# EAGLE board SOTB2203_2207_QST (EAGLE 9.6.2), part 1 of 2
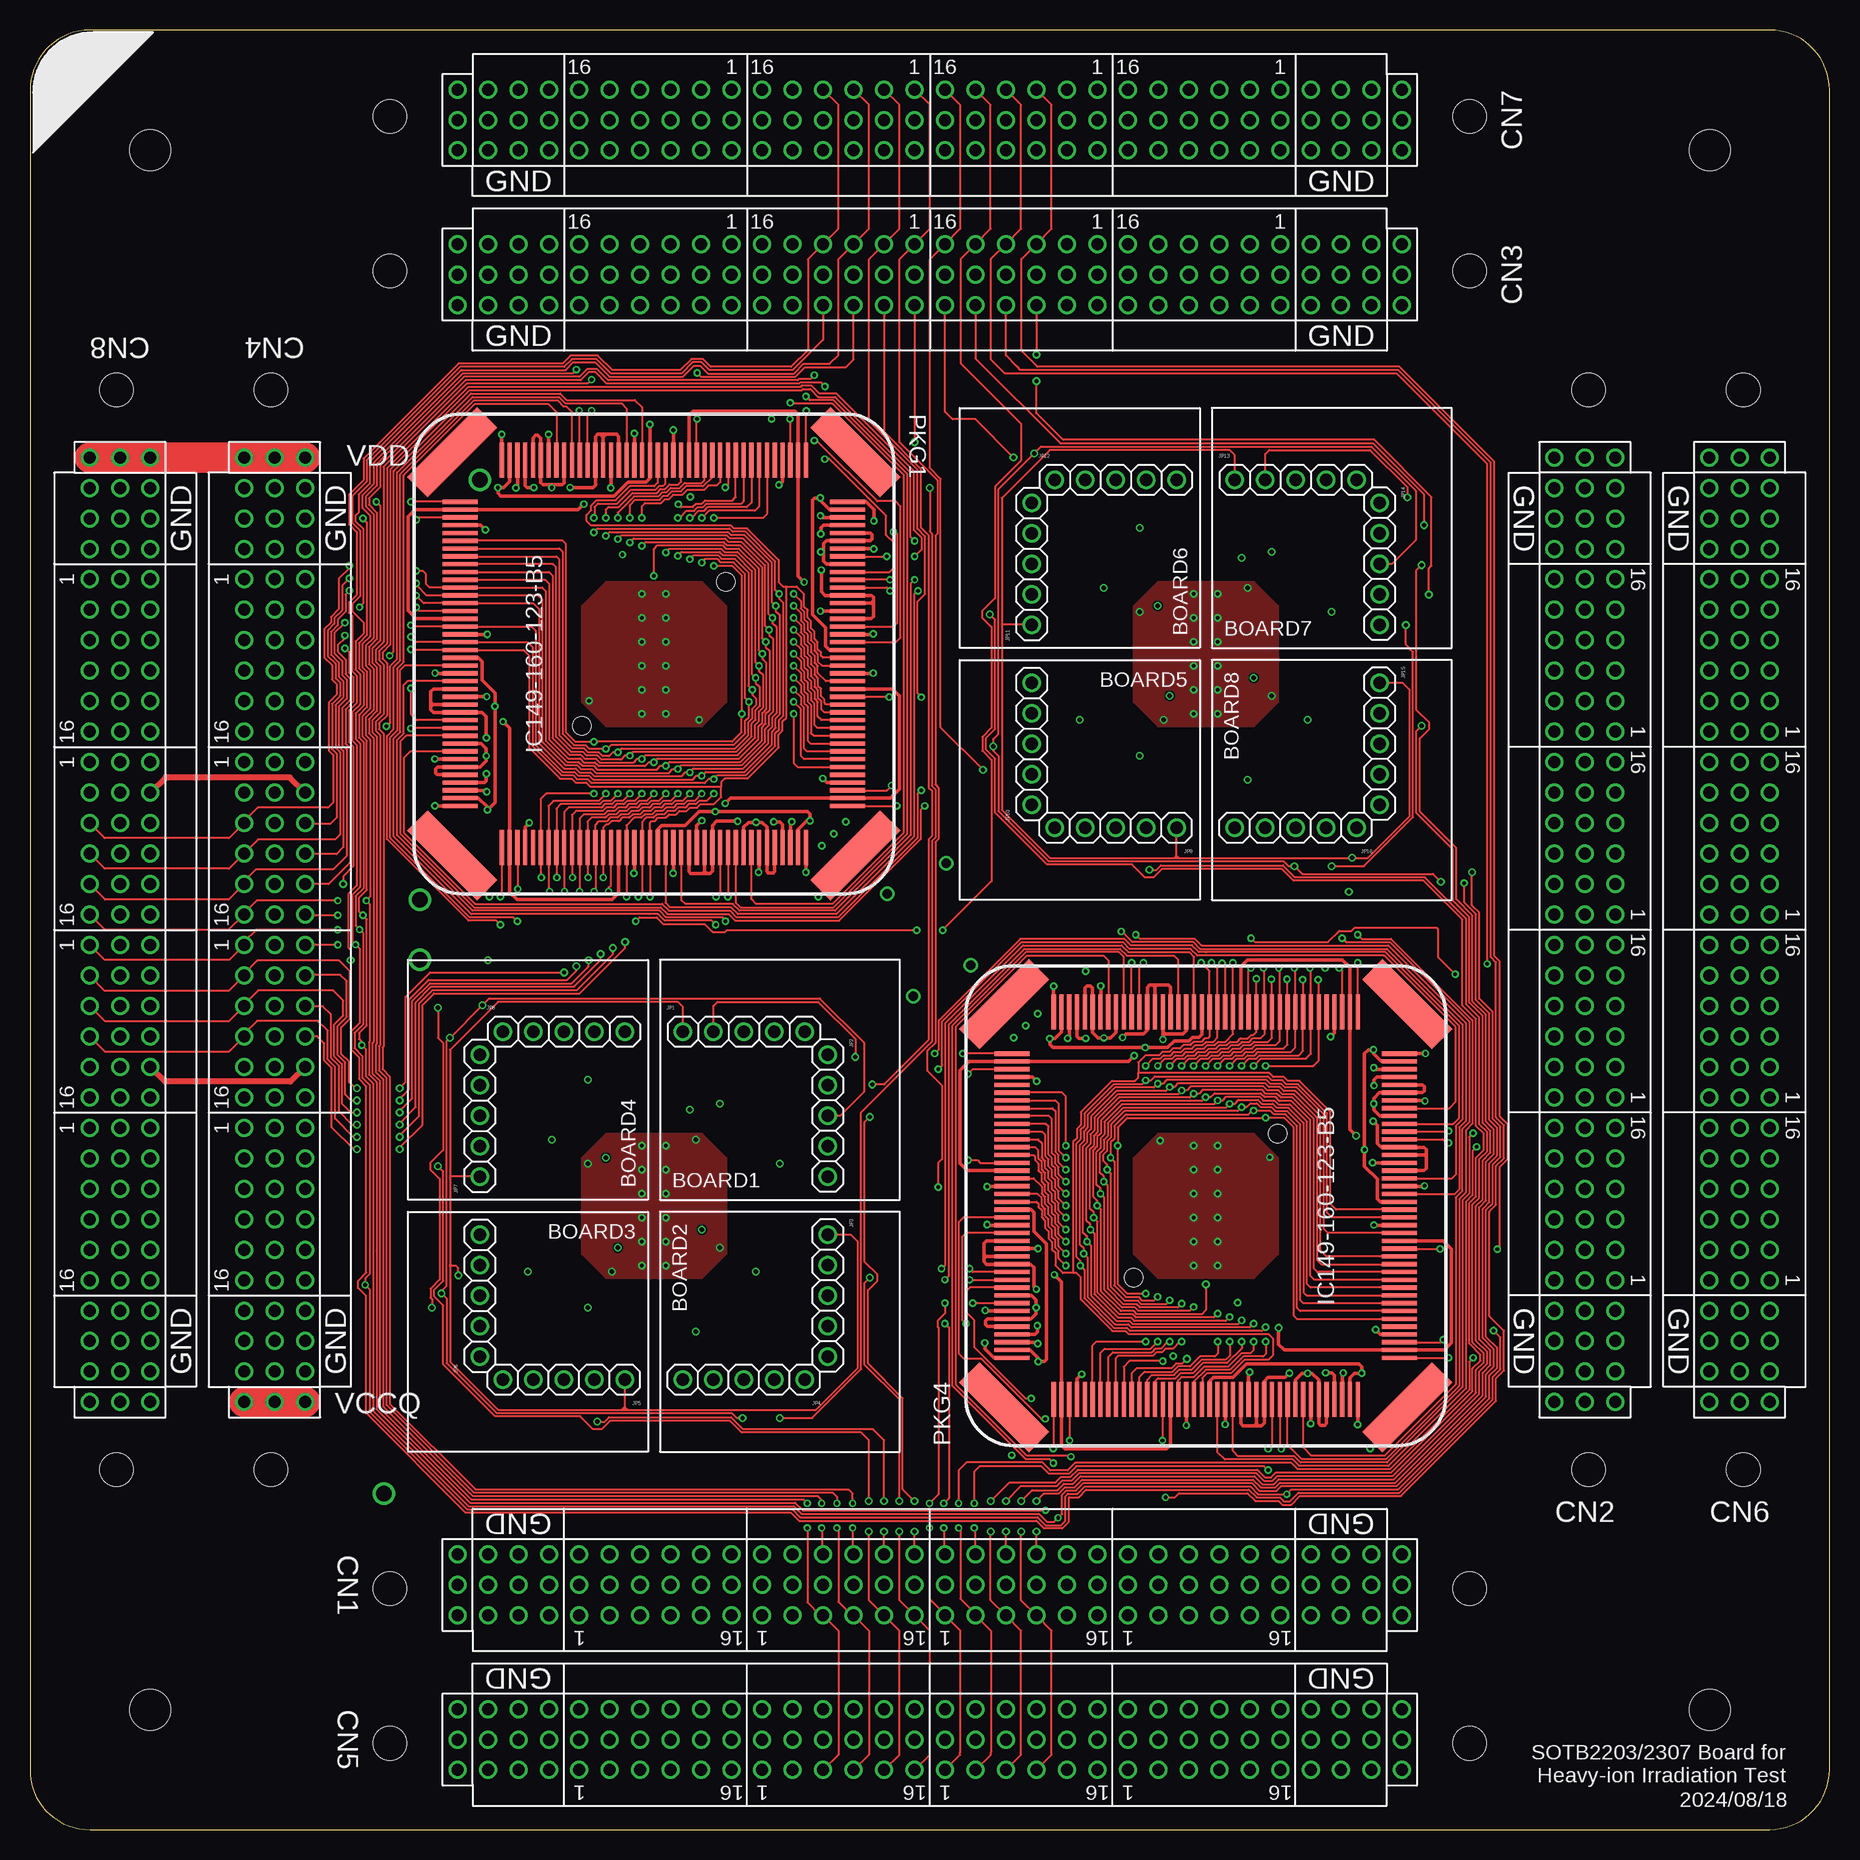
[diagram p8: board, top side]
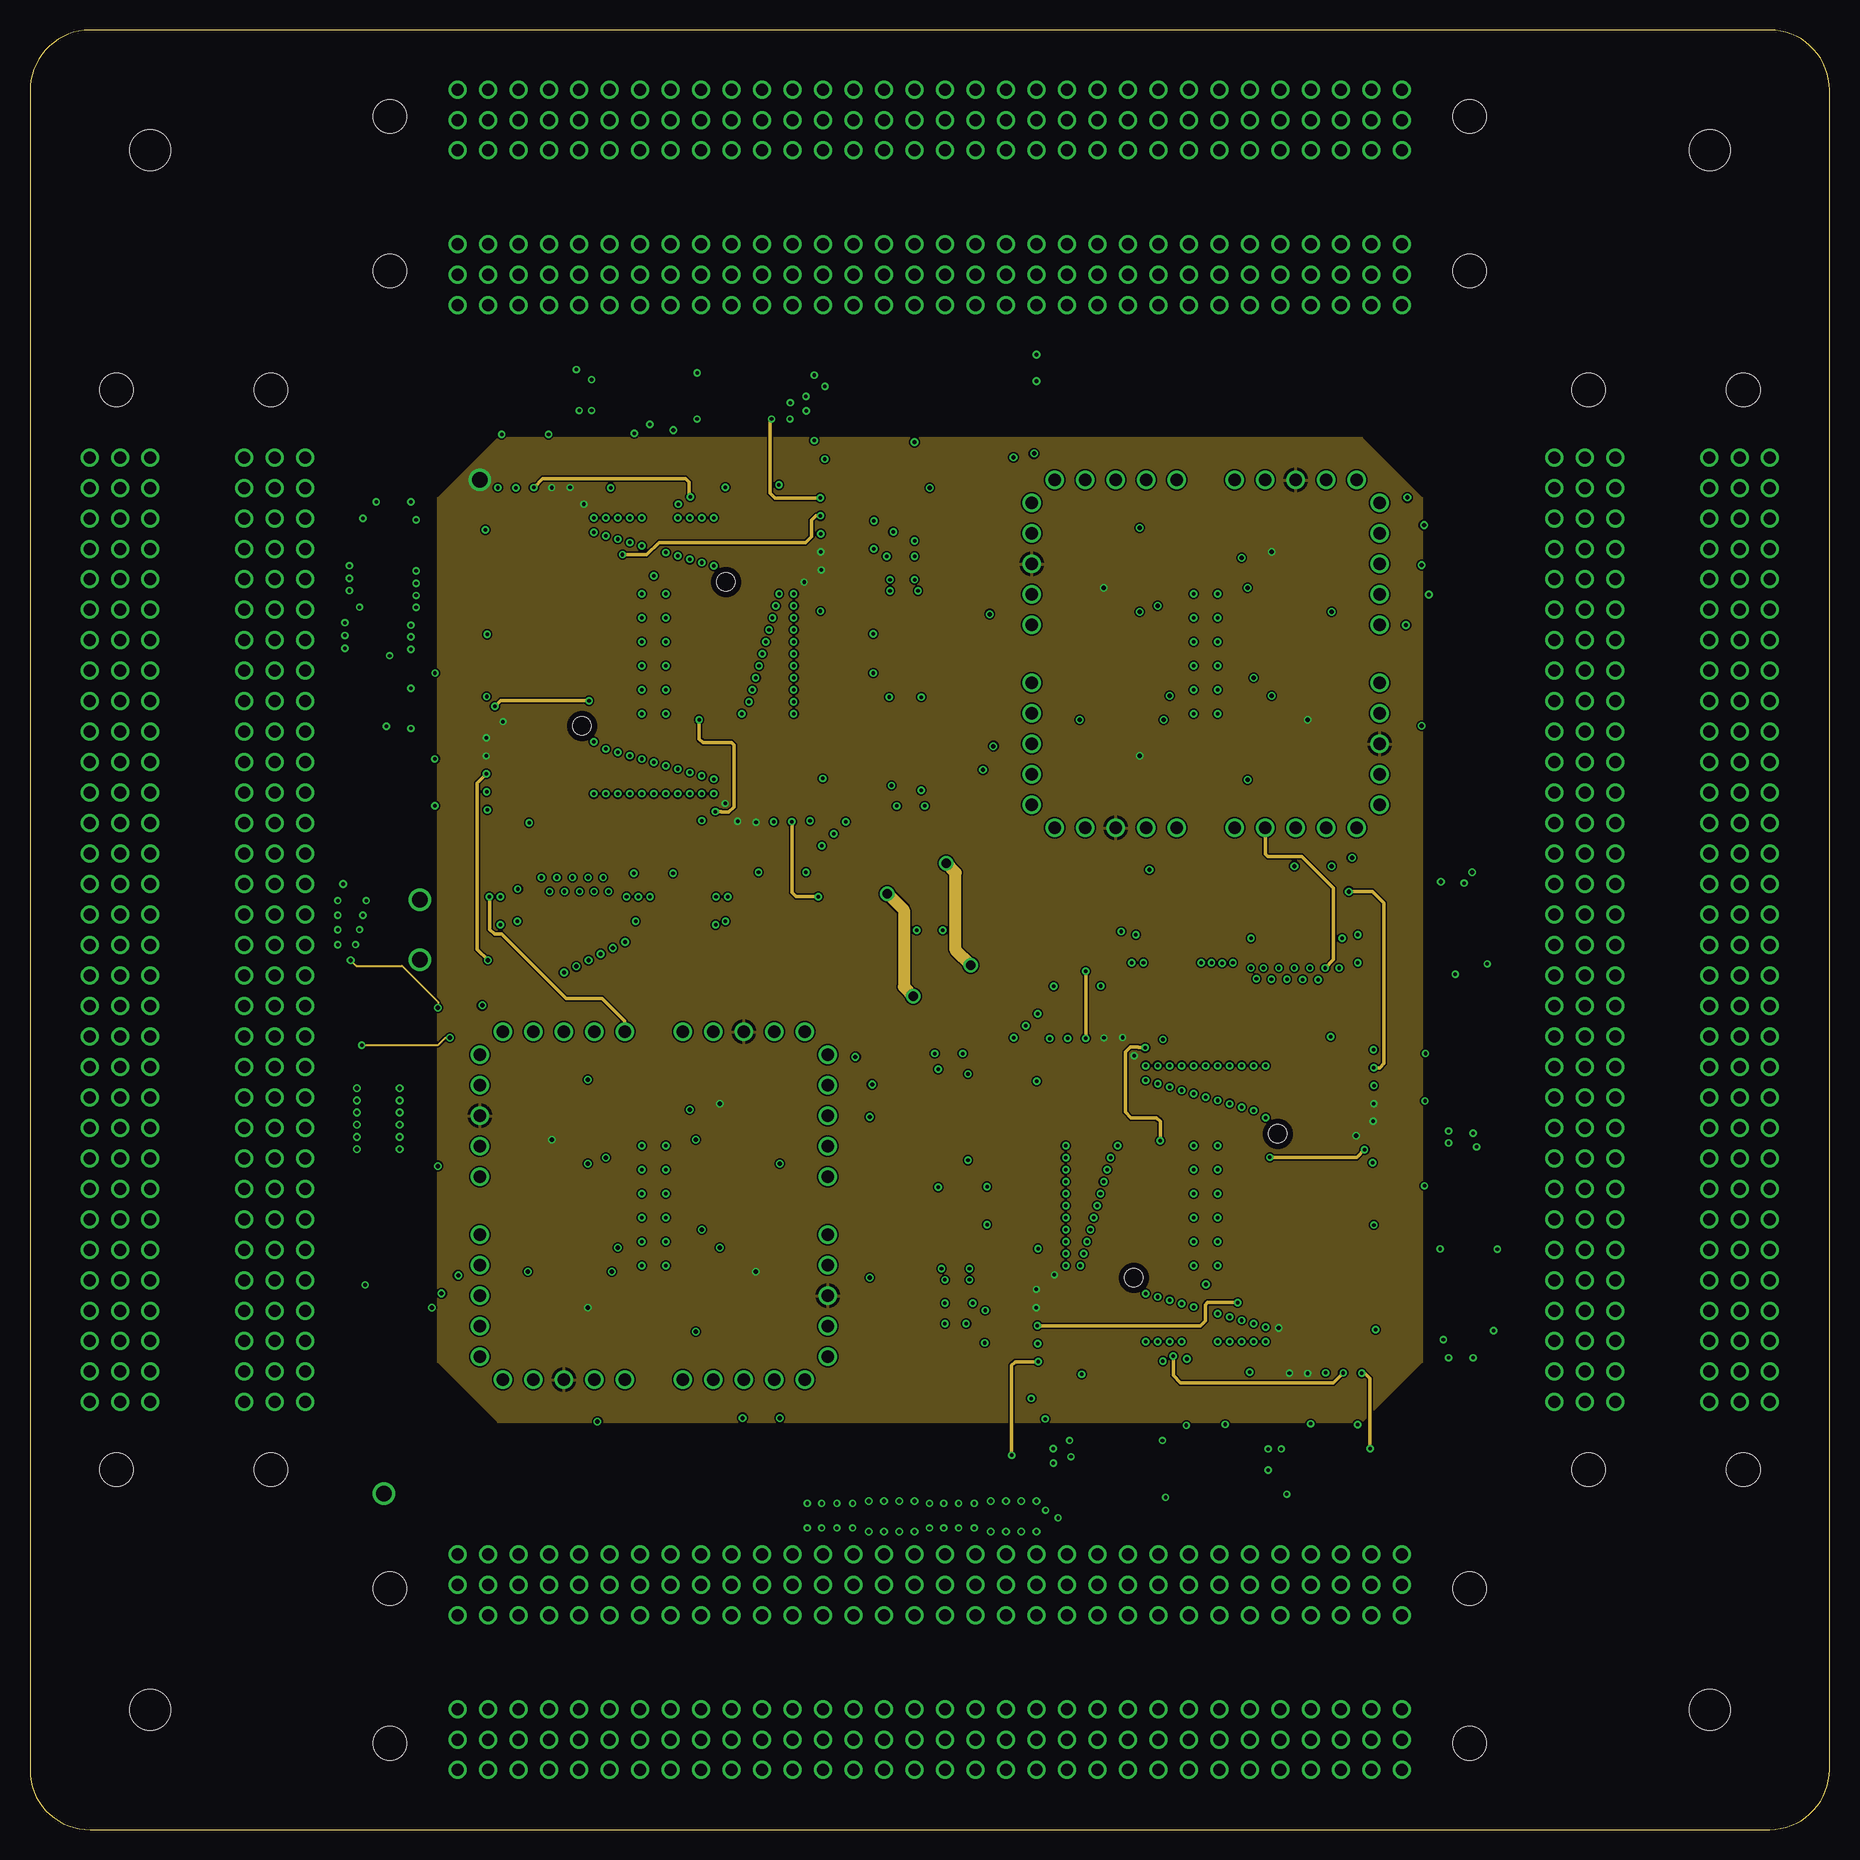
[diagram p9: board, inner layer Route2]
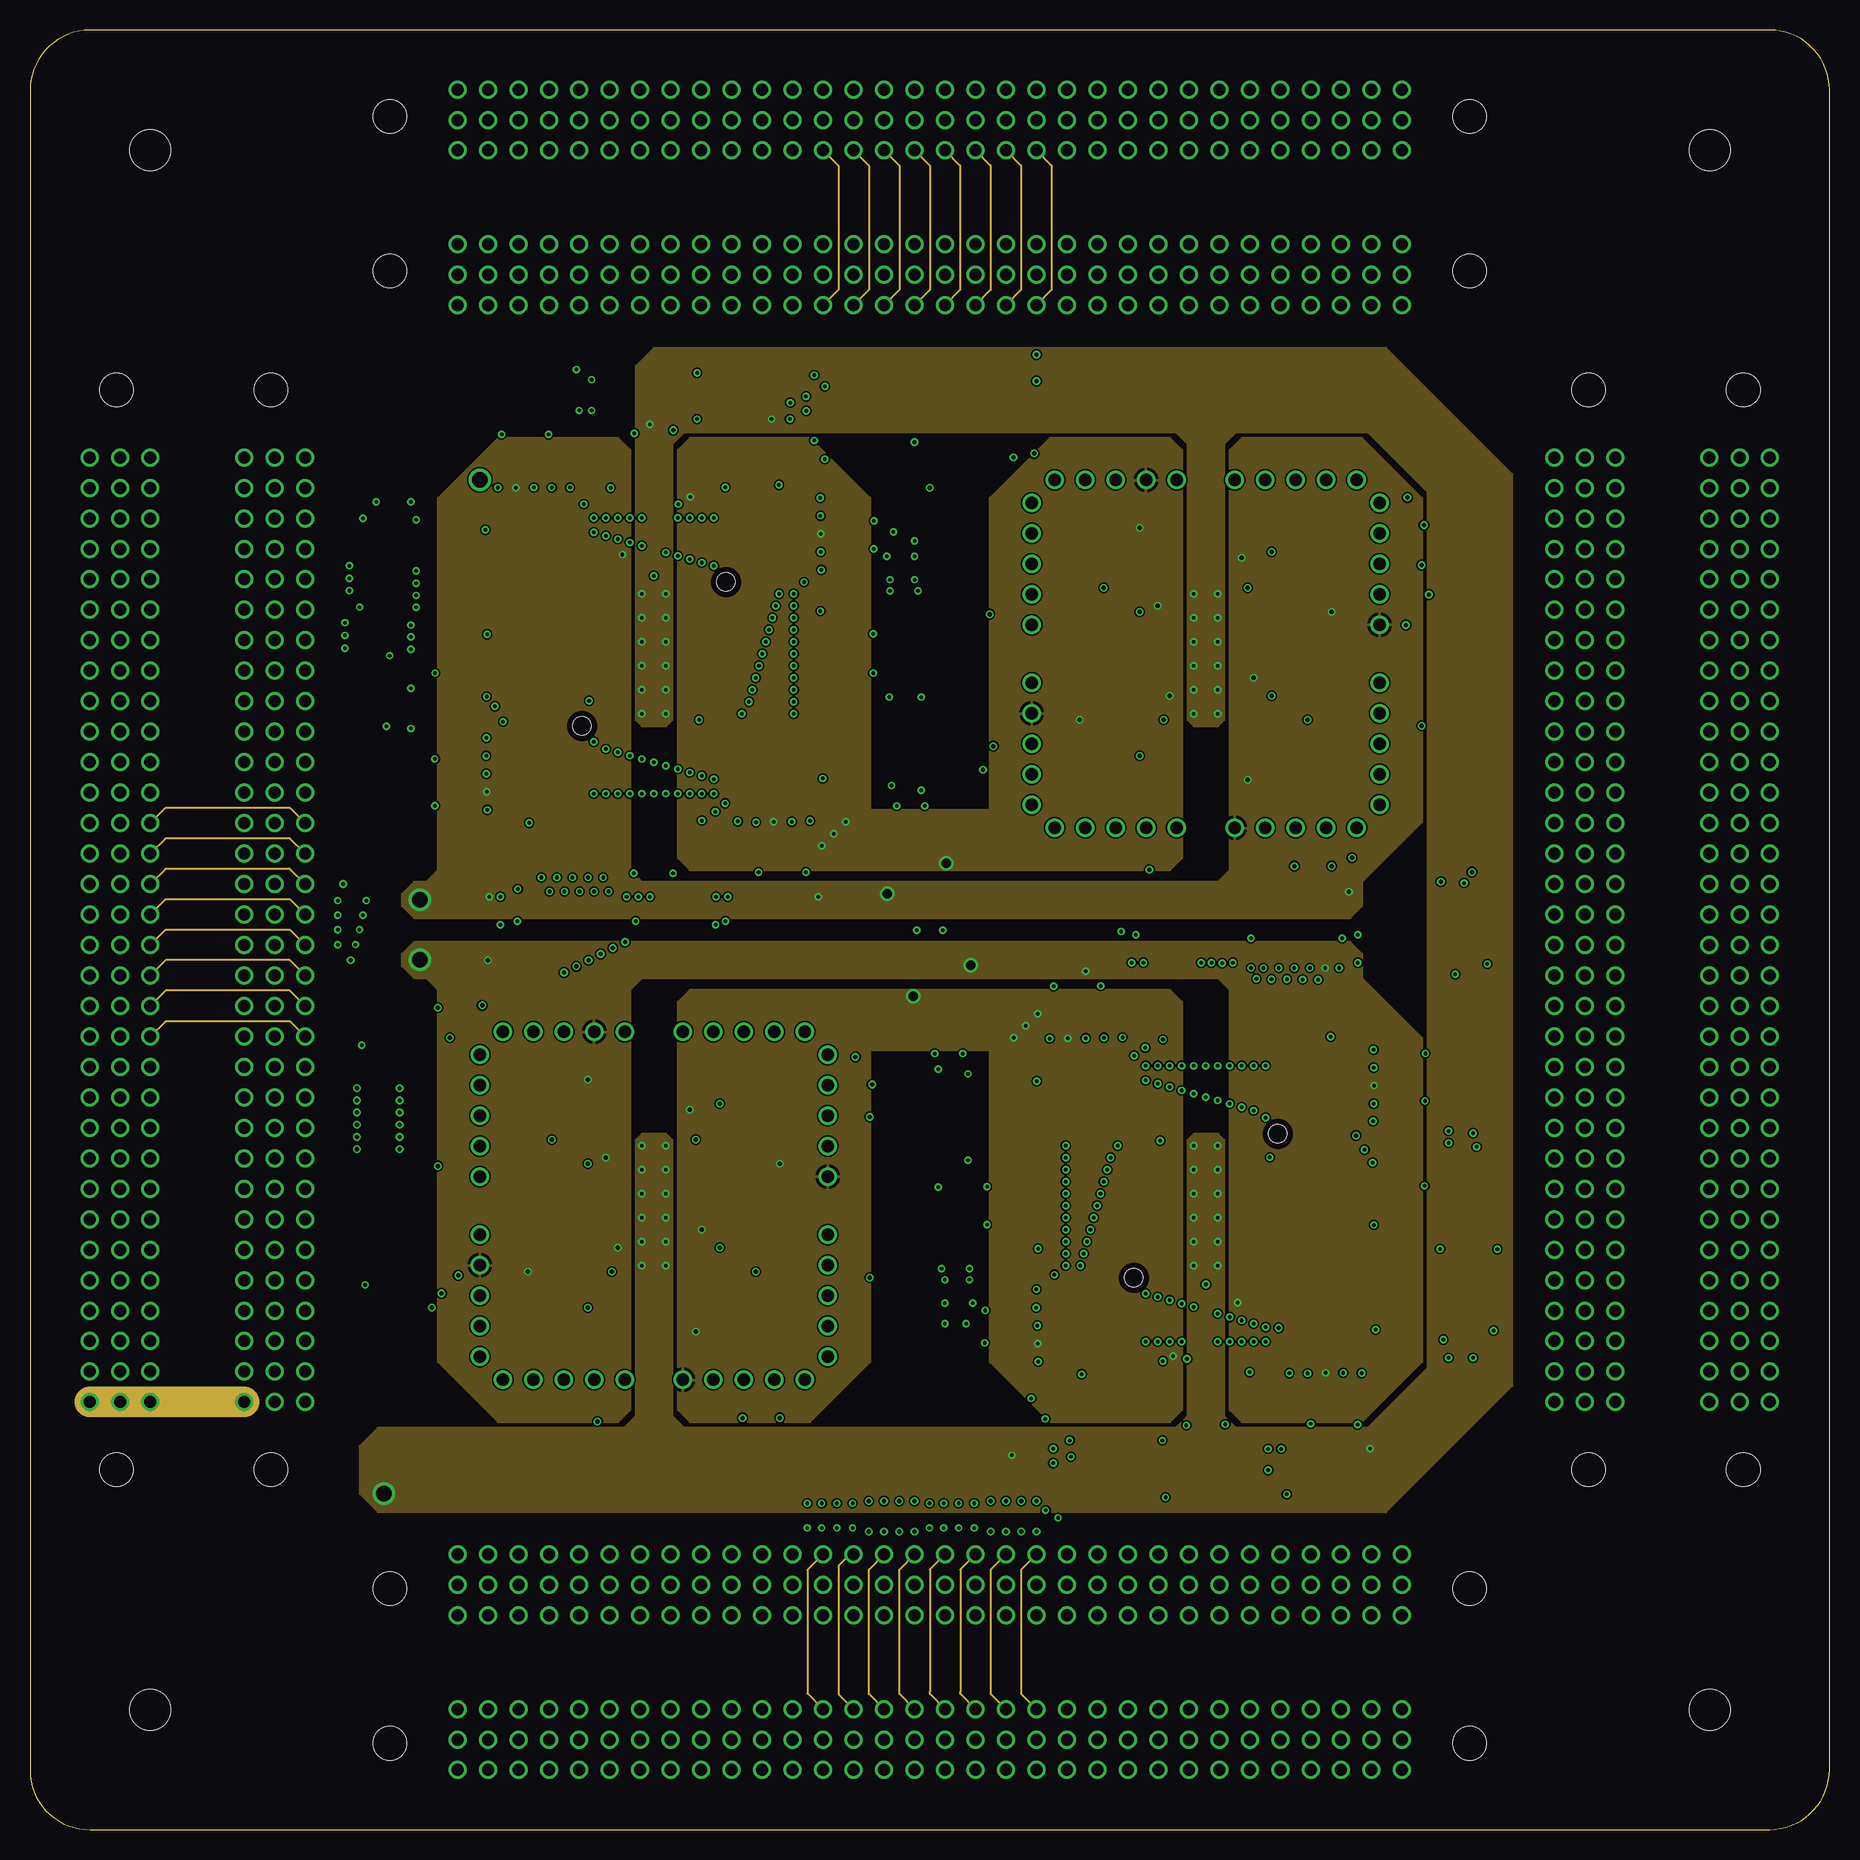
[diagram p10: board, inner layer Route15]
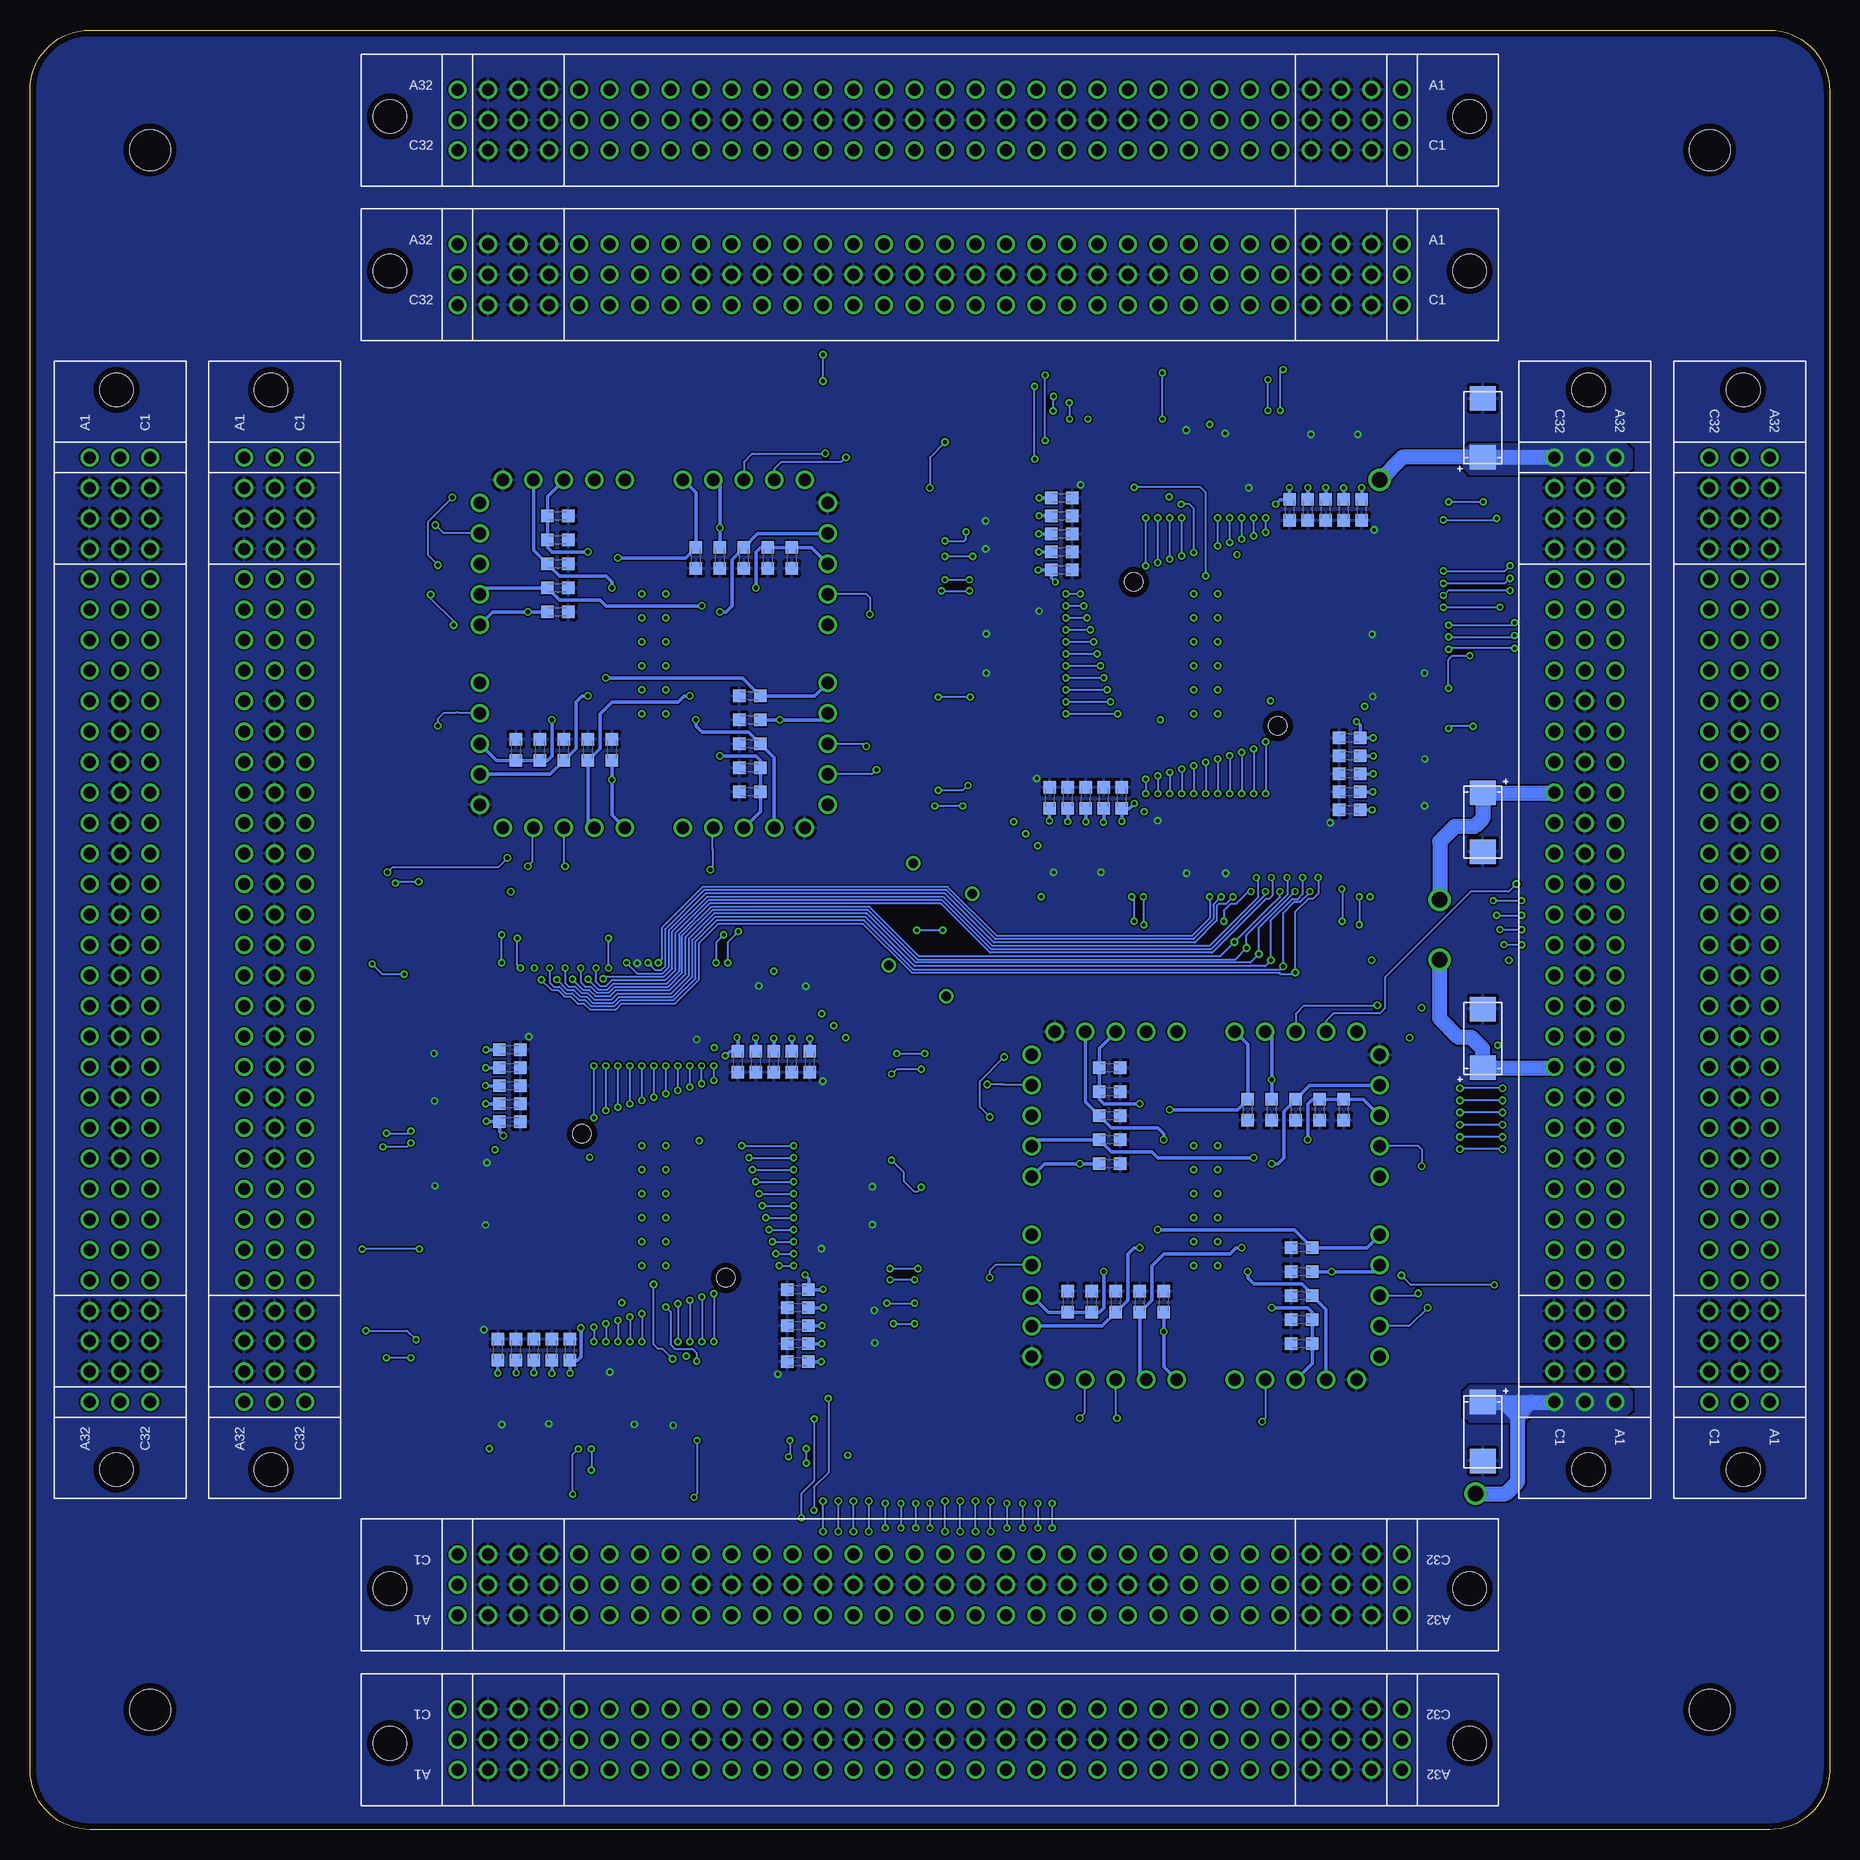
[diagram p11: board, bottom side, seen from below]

Size 150 x 150 mm. Coordinates in mm from the lower left corner, seen from the top.
Outline: 150,5 150,145 arc90 145,150 5,150 arc90 0,144.9 0,4.9 arc90 5,0 145,0 arc90 150,5
Copper layers (1+2*15+16): Top 0.018mm / dielectric 0.25mm / Route2 0.035mm / dielectric 1mm / Route15 0.035mm / dielectric 0.25mm / Bottom 0.018mm
Design rules "pban_5mil-l4": minimum track width 5mil, minimum drill 0.3mm, track to track 5mil, track to pad 0.229mm, pad to pad 5mil, via to via 5mil, smd to smd 5mil, copper to edge 0.5mm, drill to drill 0.5mm, minimum pad ring 0.15mm, minimum via ring 0.15mm, stop-mask expansion 4mil, vias tented up to drill 0.35mm, thermal gap 10mil
Holes 3.4 mm at 10,140 10,10 140,140 140,10

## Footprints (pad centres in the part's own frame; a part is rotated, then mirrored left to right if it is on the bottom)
C0603K = smd 1.05 x 1.08: 1 -0.875,0; 2 0.875,0
XC5D_9623 = drill 1: A1 39.37,2.54; A2 36.83,2.54; A3 34.29,2.54; A4 31.75,2.54; A5 29.21,2.54; A6 26.67,2.54; A7 24.13,2.54; A8 21.59,2.54; A9 19.05,2.54; A10 16.51,2.54; A11 13.97,2.54; A12 11.43,2.54; A13 8.89,2.54; A14 6.35,2.54; A15 3.81,2.54; A16 1.27,2.54; A17 -1.27,2.54; A18 -3.81,2.54; A19 -6.35,2.54; A20 -8.89,2.54; A21 -11.43,2.54; A22 -13.97,2.54; A23 -16.51,2.54; A24 -19.05,2.54; A25 -21.59,2.54; A26 -24.13,2.54; A27 -26.67,2.54; A28 -29.21,2.54; A29 -31.75,2.54; A30 -34.29,2.54; A31 -36.83,2.54; A32 -39.37,2.54; B1 39.37,0; B2 36.83,0; B3 34.29,0; B4 31.75,0; B5 29.21,0; B6 26.67,0; B7 24.13,0; B8 21.59,0; B9 19.05,0; B10 16.51,0; B11 13.97,0; B12 11.43,0; B13 8.89,0; B14 6.35,0; B15 3.81,0; B16 1.27,0; B17 -1.27,0; B18 -3.81,0; B19 -6.35,0; B20 -8.89,0; B21 -11.43,0; B22 -13.97,0; B23 -16.51,0; B24 -19.05,0; B25 -21.59,0; B26 -24.13,0; B27 -26.67,0; B28 -29.21,0; B29 -31.75,0; B30 -34.29,0; B31 -36.83,0; B32 -39.37,0; C1 39.37,-2.54; C2 36.83,-2.54; C3 34.29,-2.54; C4 31.75,-2.54; C5 29.21,-2.54; C6 26.67,-2.54; C7 24.13,-2.54; C8 21.59,-2.54; C9 19.05,-2.54; C10 16.51,-2.54; C11 13.97,-2.54; C12 11.43,-2.54; C13 8.89,-2.54; C14 6.35,-2.54; C15 3.81,-2.54; C16 1.27,-2.54; C17 -1.27,-2.54; C18 -3.81,-2.54; C19 -6.35,-2.54; C20 -8.89,-2.54; C21 -11.43,-2.54; C22 -13.97,-2.54; C23 -16.51,-2.54; C24 -19.05,-2.54; C25 -21.59,-2.54; C26 -24.13,-2.54; C27 -26.67,-2.54; C28 -29.21,-2.54; C29 -31.75,-2.54; C30 -34.29,-2.54; C31 -36.83,-2.54; C32 -39.37,-2.54 | hole 2.8: -45,0.3; 45,0.3
1X05 = drill 1.016: 1 -5.08,0; 2 -2.54,0; 3 0,0; 4 2.54,0; 5 5.08,0
IC149-160-123-B5 = smd 0.35 x 2.9: 1 -12.675,-16.15; 2 -12.025,-16.15; 3 -11.375,-16.15; 4 -10.725,-16.15; 5 -10.075,-16.15; 6 -9.425,-16.15; 7 -8.775,-16.15; 8 -8.125,-16.15; 9 -7.475,-16.15; 10 -6.825,-16.15; 11 -6.175,-16.15; 12 -5.525,-16.15; 13 -4.875,-16.15; 14 -4.225,-16.15; 15 -3.575,-16.15; 16 -2.925,-16.15; 17 -2.275,-16.15; 18 -1.625,-16.15; 19 -0.975,-16.15; 20 -0.325,-16.15; 21 0.325,-16.15; 22 0.975,-16.15; 23 1.625,-16.15; 24 2.275,-16.15; 25 2.925,-16.15; 26 3.575,-16.15; 27 4.225,-16.15; 28 4.875,-16.15; 29 5.525,-16.15; 30 6.175,-16.15; 31 6.825,-16.15; 32 7.475,-16.15; 33 8.125,-16.15; 34 8.775,-16.15; 35 9.425,-16.15; 36 10.075,-16.15; 37 10.725,-16.15; 38 11.375,-16.15; 39 12.025,-16.15; 40 12.675,-16.15; 81 12.675,16.15; 82 12.025,16.15; 83 11.375,16.15; 84 10.725,16.15; 85 10.075,16.15; 86 9.425,16.15; 87 8.775,16.15; 88 8.125,16.15; 89 7.475,16.15; 90 6.825,16.15; 91 6.175,16.15; 92 5.525,16.15; 93 4.875,16.15; 94 4.225,16.15; 95 3.575,16.15; 96 2.925,16.15; 97 2.275,16.15; 98 1.625,16.15; 99 0.975,16.15; 100 0.325,16.15; 101 -0.325,16.15; 102 -0.975,16.15; 103 -1.625,16.15; 104 -2.275,16.15; 105 -2.925,16.15; 106 -3.575,16.15; 107 -4.225,16.15; 108 -4.875,16.15; 109 -5.525,16.15; 110 -6.175,16.15; 111 -6.825,16.15; 112 -7.475,16.15; 113 -8.125,16.15; 114 -8.775,16.15; 115 -9.425,16.15; 116 -10.075,16.15; 117 -10.725,16.15; 118 -11.375,16.15; 119 -12.025,16.15; 120 -12.675,16.15 | smd 2.9 x 0.35: 41 16.15,-12.675; 42 16.15,-12.025; 43 16.15,-11.375; 44 16.15,-10.725; 45 16.15,-10.075; 46 16.15,-9.425; 47 16.15,-8.775; 48 16.15,-8.125; 49 16.15,-7.475; 50 16.15,-6.825; 51 16.15,-6.175; 52 16.15,-5.525; 53 16.15,-4.875; 54 16.15,-4.225; 55 16.15,-3.575; 56 16.15,-2.925; 57 16.15,-2.275; 58 16.15,-1.625; 59 16.15,-0.975; 60 16.15,-0.325; 61 16.15,0.325; 62 16.15,0.975; 63 16.15,1.625; 64 16.15,2.275; 65 16.15,2.925; 66 16.15,3.575; 67 16.15,4.225; 68 16.15,4.875; 69 16.15,5.525; 70 16.15,6.175; 71 16.15,6.825; 72 16.15,7.475; 73 16.15,8.125; 74 16.15,8.775; 75 16.15,9.425; 76 16.15,10.075; 77 16.15,10.725; 78 16.15,11.375; 79 16.15,12.025; 80 16.15,12.675; 121 -16.15,12.675; 122 -16.15,12.025; 123 -16.15,11.375; 124 -16.15,10.725; 125 -16.15,10.075; 126 -16.15,9.425; 127 -16.15,8.775; 128 -16.15,8.125; 129 -16.15,7.475; 130 -16.15,6.825; 131 -16.15,6.175; 132 -16.15,5.525; 133 -16.15,4.875; 134 -16.15,4.225; 135 -16.15,3.575; 136 -16.15,2.925; 137 -16.15,2.275; 138 -16.15,1.625; 139 -16.15,0.975; 140 -16.15,0.325; 141 -16.15,-0.325; 142 -16.15,-0.975; 143 -16.15,-1.625; 144 -16.15,-2.275; 145 -16.15,-2.925; 146 -16.15,-3.575; 147 -16.15,-4.225; 148 -16.15,-4.875; 149 -16.15,-5.525; 150 -16.15,-6.175; 151 -16.15,-6.825; 152 -16.15,-7.475; 153 -16.15,-8.125; 154 -16.15,-8.775; 155 -16.15,-9.425; 156 -16.15,-10.075; 157 -16.15,-10.725; 158 -16.15,-11.375; 159 -16.15,-12.025; 160 -16.15,-12.675 | smd 8.2 x 2.4 rotated 315: M1 -16.8,-16.8; M3 16.8,16.8 | smd 8.2 x 2.4 rotated 45: M2 16.8,-16.8; M4 -16.8,16.8 | hole 1.5: -6,6; 6,-6
6032 = smd 2.032 x 2.2: + 0.55,-1.6; - 5.45,-1.6

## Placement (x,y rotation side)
C1  [C0603K]  40,91 180 bottom
C2  [C0603K]  40,89.5 180 bottom
C3  [C0603K]  40,85 180 bottom
C4  [C0603K]  40,88 180 bottom
C5  [C0603K]  40,86.5 180 bottom
C6  [C0603K]  59,86 90 bottom
C7  [C0603K]  60.5,86 90 bottom
C8  [C0603K]  65,86 90 bottom
C9  [C0603K]  62,86 90 bottom
C10  [C0603K]  63.5,86 90 bottom
C11  [C0603K]  64,105 0 bottom
C12  [C0603K]  64,106.5 0 bottom
C13  [C0603K]  64,111 0 bottom
C14  [C0603K]  64,108 0 bottom
C15  [C0603K]  64,109.5 0 bottom
C16  [C0603K]  45,110 270 bottom
C17  [C0603K]  43.5,110 270 bottom
C18  [C0603K]  39,110 270 bottom
C19  [C0603K]  42,110 270 bottom
C20  [C0603K]  40.5,110 270 bottom
C21  [C0603K]  63.5,44 90 bottom
C22  [C0603K]  61.5,44 90 bottom
C23  [C0603K]  59.5,44 90 bottom
C24  [C0603K]  57.5,44 90 bottom
C25  [C0603K]  55.5,44 90 bottom
C26  [C0603K]  60,63.5 0 bottom
C27  [C0603K]  60,61.5 0 bottom
C28  [C0603K]  60,59.5 0 bottom
C29  [C0603K]  60,57.5 0 bottom
C30  [C0603K]  60,55.5 0 bottom
C31  [C0603K]  40.5,60 270 bottom
C32  [C0603K]  42.5,60 270 bottom
C33  [C0603K]  44.5,60 270 bottom
C34  [C0603K]  46.5,60 270 bottom
C35  [C0603K]  48.5,60 270 bottom
C36  [C0603K]  44,40.5 180 bottom
C37  [C0603K]  44,42.5 180 bottom
C38  [C0603K]  44,44.5 180 bottom
C39  [C0603K]  44,46.5 180 bottom
C40  [C0603K]  44,48.5 180 bottom
C41  [C0603K]  86.5,106 270 bottom
C42  [C0603K]  88.5,106 270 bottom
C43  [C0603K]  90.5,106 270 bottom
C44  [C0603K]  92.5,106 270 bottom
C45  [C0603K]  94.5,106 270 bottom
C46  [C0603K]  90,86.5 180 bottom
C47  [C0603K]  90,88.5 180 bottom
C48  [C0603K]  90,90.5 180 bottom
C49  [C0603K]  90,92.5 180 bottom
C50  [C0603K]  90,94.5 180 bottom
C51  [C0603K]  109.5,90 90 bottom
C52  [C0603K]  107.5,90 90 bottom
C53  [C0603K]  105.5,90 90 bottom
C54  [C0603K]  103.5,90 90 bottom
C55  [C0603K]  101.5,90 90 bottom
C56  [C0603K]  106,109.5 0 bottom
C57  [C0603K]  106,107.5 0 bottom
C58  [C0603K]  106,105.5 0 bottom
C59  [C0603K]  106,103.5 0 bottom
C60  [C0603K]  106,101.5 0 bottom
C61  [C0603K]  110,59 0 bottom
C62  [C0603K]  110,60.5 0 bottom
C63  [C0603K]  110,65 0 bottom
C64  [C0603K]  110,62 0 bottom
C65  [C0603K]  110,63.5 0 bottom
C66  [C0603K]  91,64 270 bottom
C67  [C0603K]  89.5,64 270 bottom
C68  [C0603K]  85,64 270 bottom
C69  [C0603K]  88,64 270 bottom
C70  [C0603K]  86.5,64 270 bottom
C71  [C0603K]  86,45 180 bottom
C72  [C0603K]  86,43.5 180 bottom
C73  [C0603K]  86,39 180 bottom
C74  [C0603K]  86,42 180 bottom
C75  [C0603K]  86,40.5 180 bottom
C76  [C0603K]  105,40 90 bottom
C77  [C0603K]  106.5,40 90 bottom
C78  [C0603K]  111,40 90 bottom
C79  [C0603K]  108,40 90 bottom
C80  [C0603K]  109.5,40 90 bottom
CN1  XC5G-9621  [XC5D_9623]  75,20.39 180 bottom
CN2  XC5G-9621  [XC5D_9623]  129.61,75 90 bottom
CN3  XC5G-9621  [XC5D_9623]  75,129.61 0 bottom
CN4  XC5G-9621  [XC5D_9623]  20.39,75 270 bottom
CN5  XC5G-9621  [XC5D_9623]  75,7.5 180 bottom
CN6  XC5G-9621  [XC5D_9623]  142.5,75 90 bottom
CN7  XC5G-9621  [XC5D_9623]  75,142.5 0 bottom
CN8  XC5G-9621  [XC5D_9623]  7.5,75 270 bottom
JP1  [1X05]  59.5,66.5 0 top
JP2  [1X05]  66.5,59.5 270 top
JP3  [1X05]  66.5,44.5 270 top
JP4  [1X05]  59.5,37.5 180 top
JP5  [1X05]  44.5,37.5 180 top
JP6  [1X05]  37.5,44.5 90 top
JP7  [1X05]  37.5,59.5 90 top
JP8  [1X05]  44.5,66.5 0 top
JP9  [1X05]  90.5,83.5 180 top
JP10  [1X05]  83.5,90.5 90 top
JP11  [1X05]  83.5,105.5 90 top
JP12  [1X05]  90.5,112.5 0 top
JP13  [1X05]  105.5,112.5 0 top
JP14  [1X05]  112.5,105.5 270 top
JP15  [1X05]  112.5,90.5 270 top
JP16  [1X05]  105.5,83.5 180 top
PKG1  SOTB2207_4CHIP  [IC149-160-123-B5]  52,98 270 top
PKG4  SOTB2207_4CHIP  [IC149-160-123-B5]  98,52 90 top
U$5  TANTALUM_CAPA_F93  [6032]  30.5,113.84 90 bottom
U$6  TANTALUM_CAPA_F93  [6032]  27.3,36.16 270 bottom
U$7  TANTALUM_CAPA_F93  [6032]  30.5,62.94 90 bottom
U$8  TANTALUM_CAPA_F93  [6032]  27.3,86.96 270 bottom

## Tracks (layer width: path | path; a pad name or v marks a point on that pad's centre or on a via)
A_ENCLKIN  (via drill 0.3)
  Top 0.152: PKG4.17 108.19,49.73 107.84,50.07 107.84,59.59 105.59,61.84 104.62,61.84 104.3,62.17 103.39,62.17 103.06,62.49 94.75,62.49 94.42,62.17 v94.01,62.17 93.68,61.84 90.43,61.84 88.16,59.57 88.16,58.5 87.83,58.18 87.83,57.39 87.51,57.06 87.51,48.75 87.83,48.42 v87.83,48 88.16,47.67 88.16,44.41 90.46,42.11 91.55,42.11 91.82,41.83 101.67,41.83 v102,42.16 | v86.34,48 85.74,48.61 85.74,49.21 85.46,49.49 85.46,50.09 85.18,50.37 85.18,50.98 84.9,51.26 84.9,51.86 84.62,52.14 84.62,52.75 84.34,53.03 84.34,53.6 83.67,54.27 PKG4.97 | v94.01,63.66 94.61,64.26 95.21,64.26 95.49,64.54 96.09,64.54 96.37,64.82 96.98,64.82 97.26,65.1 97.86,65.1 98.14,65.38 98.75,65.38 99.03,65.66 99.63,65.66 100.28,66.3 PKG4.57 v100.28,72.25 v100.27,72.25 | v63.66,102 64.26,101.39 64.26,100.79 64.54,100.51 64.54,99.91 64.82,99.63 64.82,99.02 65.1,98.74 65.1,98.14 65.38,97.86 65.38,97.25 65.66,96.97 65.66,96.4 66.33,95.72 PKG1.97 | v55.99,86.34 55.39,85.74 54.79,85.74 54.51,85.46 53.91,85.46 53.63,85.18 53.02,85.18 52.74,84.9 52.14,84.9 51.86,84.62 51.25,84.62 50.97,84.34 50.37,84.34 49.73,83.7 PKG1.57 v49.73,77.75 | v48,107.84 48.33,108.17 58.18,108.17 58.45,107.89 59.54,107.89 61.84,105.59 61.84,102.33 v62.17,102 62.17,101.58 62.49,101.25 62.49,92.94 62.17,92.61 62.17,91.82 61.84,91.5 61.84,90.43 59.57,88.16 56.32,88.16 v55.99,87.83 55.58,87.83 55.25,87.51 46.94,87.51 46.61,87.83 45.7,87.83 45.38,88.16 44.41,88.16 42.16,90.41 42.16,99.93 41.81,100.28 PKG1.17 31.86,100.28 v31.75,100.38 | v26.26,100.6 25.37,99.72 25.37,98.05 26.02,97.4 26.02,96.21 26.4,95.84 26.4,94.25 25.75,93.6 25.75,90.29 26.12,89.92 26.12,81.88 25.55,81.31 22.97,81.31 CN4.C19
  Top 0.152: PKG4.137 95.72,37.45 96.02,37.75 97.04,37.75 97.89,38.6 99.89,38.6 101.01,39.71 101.75,39.71 102,39.96 v102,40.67 | v48,109.33 48,110.03 48.21,110.24 49.06,110.24 50.22,111.4 52.25,111.4 52.58,111.73 52.92,111.73 53.3,112.11 54.04,112.11 54.27,112.34 PKG1.137
  Route15 0.152: CN4.C19 21.66,82.62 11.31,82.62 CN8.C19
  Bottom 0.152: v87.83,48 v86.34,48 | v94.01,62.17 v94.01,63.66 | v102,42.16 v102,40.67 | v62.17,102 v63.66,102 | v55.99,87.83 v55.99,86.34 | v48,107.84 v48,109.33 | v49.73,77.75 50.33,77.15 50.92,77.15 51.09,76.98 51.09,75.76 52.91,73.93 69.64,73.93 73.73,78.02 93.69,78.02 96.75,74.96 96.75,71.88 97.26,71.36 99.39,71.36 v100.27,72.25 | v31.75,100.38 26.47,100.38 v26.26,100.6
A_ENCNTIN  (via drill 0.3, 0.35)
  Top 0.152: PKG4.11 107.06,45.83 106.72,46.16 106.72,59.13 105.13,60.72 104.16,60.72 103.83,61.05 102.92,61.05 102.6,61.38 98.75,61.38 98.42,61.05 v98,61.05 97.67,60.72 90.89,60.72 89.28,59.11 89.28,58.04 88.95,57.71 88.95,56.92 88.62,56.6 88.62,52.75 88.95,52.42 v88.95,52 89.28,51.67 89.28,44.87 90.92,43.23 92.01,43.23 92.29,42.95 97.67,42.95 98.02,43.3 v98.02,45.44 | v86.34,52 85.74,52.61 85.74,53.21 85.46,53.49 85.46,54.09 85.18,54.37 85.18,54.98 84.9,55.26 84.9,55.86 84.62,56.14 84.62,57.92 84.36,58.17 PKG4.91 | v98,63.66 98.61,64.26 99.21,64.26 99.49,64.54 100.09,64.54 100.37,64.82 100.98,64.82 101.26,65.1 101.86,65.1 102.14,65.38 103.84,65.38 104.17,65.72 PKG4.51 104.17,71.73 v104.09,71.82 | PKG1.11 42.95,104.17 43.28,103.84 43.28,90.87 44.87,89.28 45.84,89.28 46.17,88.95 47.08,88.95 47.4,88.62 51.25,88.62 51.58,88.95 v52,88.95 52.33,89.28 59.11,89.28 60.72,90.89 60.72,91.96 61.05,92.29 61.05,93.08 61.38,93.4 61.38,97.25 61.05,97.58 v61.05,98 60.72,98.33 60.72,105.13 59.08,106.77 57.99,106.77 57.71,107.05 52.33,107.05 52,106.72 v52,104.5 | v63.66,98 64.26,97.39 64.26,96.79 64.54,96.51 64.54,95.91 64.82,95.63 64.82,95.02 65.1,94.74 65.1,94.14 65.38,93.86 65.38,92.08 65.64,91.83 PKG1.91 | v52,86.34 51.39,85.74 50.79,85.74 50.51,85.46 49.91,85.46 49.63,85.18 49.02,85.18 48.74,84.9 48.14,84.9 47.86,84.62 46.16,84.62 45.83,84.28 PKG1.51 45.83,78.2 v45.81,78.18 | PKG4.131 91.83,38.02 92.24,38.44 95.13,38.44 95.56,38.87 96.08,38.87 v96.43,39.22 | PKG1.131 58.17,112.1 v57.96,111.88 | CN4.C13 23.95,66.11 24.53,65.53 24.53,64.09 25.16,63.47 25.16,58.53 26.98,56.71 v27.25,56.71
  Top 0.152: v30.8,56.71 30.8,56.84 32.71,58.74 32.71,68.72 33.69,69.7 45.82,69.7 49.6,73.48 v49.6,73.98
  Route15 0.152: CN4.C13 21.67,67.37 11.3,67.37 CN8.C13
  Bottom 0.152: v88.95,52 v86.34,52 | v98,61.05 v98,63.66 | v61.05,98 v63.66,98 | v52,88.95 v52,86.34 | v104.09,71.82 104.09,70.63 103.73,70.27 103.27,70.27 102.75,69.75 101.74,69.75 101.25,70.25 96.8,70.25 95.63,71.42 95.63,74.5 93.22,76.91 80.01,76.91 75.92,72.82 50.77,72.82 v49.6,73.98 46.28,77.3 46.23,77.3 45.81,77.72 v45.81,78.18 | v96.43,39.22 97.28,40.06 97.63,40.06 98.01,40.44 v98.01,45.43 v98.02,45.44 | v57.96,111.88 52.44,111.88 52,111.44 v52,104.5 | v27.25,56.71 v30.8,56.71
A_ENRSTIN  (via drill 0.3, 0.35)
  Top 0.152: PKG4.8 106.12,43.88 105.89,44.11 105.89,58.78 104.78,59.88 103.81,59.88 103.49,60.21 102.58,60.21 102.25,60.54 101.75,60.54 101.42,60.21 v101,60.21 100.67,59.88 91.24,59.88 90.11,58.76 90.11,57.69 89.79,57.37 89.79,56.58 89.46,56.25 89.46,55.75 89.79,55.42 v89.79,55 90.11,54.67 90.11,45.22 91.27,44.07 92.36,44.07 92.63,43.79 94.67,43.79 v95,44.11 | v86.34,55 85.74,55.61 85.74,56.21 85.46,56.49 85.46,59.9 85.23,60.12 PKG4.88 | v101,63.66 101.61,64.26 102.21,64.26 102.49,64.54 105.75,64.54 106.12,64.91 PKG4.48 106.12,70.8 v106.08,70.84 | v95,40.67 94.86,40.67 94.25,40.06 93.79,40.06 93.51,39.78 90.27,39.78 89.88,39.4 PKG4.128 | PKG1.8 43.88,106.12 44.11,105.89 44.11,91.22 45.22,90.11 46.19,90.11 46.51,89.79 47.42,89.79 47.75,89.46 48.25,89.46 48.58,89.79 v49,89.79 49.33,90.11 58.76,90.11 59.88,91.24 59.88,92.31 60.21,92.63 60.21,93.42 60.54,93.75 60.54,94.25 60.21,94.58 v60.21,95 59.88,95.33 59.88,104.78 58.73,105.93 57.64,105.93 57.37,106.21 55.33,106.21 v55,105.89 | v63.66,95 64.26,94.39 64.26,93.79 64.54,93.51 64.54,90.1 64.77,89.88 PKG1.88 | v49,86.34 48.39,85.74 47.79,85.74 47.51,85.46 44.25,85.46 43.88,85.09 PKG1.48 43.88,79.4 v43.92,79.35 | v55,109.33 55.14,109.33 55.75,109.94 56.21,109.94 56.49,110.22 59.73,110.22 60.12,110.6 PKG1.128 | CN8.A14 6.25,67.36 16.56,67.36 CN4.A14 17.85,68.78 19.01,69.94 25.28,69.94 26.12,69.1 26.12,67.85 25.37,67.11 25.37,64.43 25.99,63.81 25.99,60.52 26.75,59.76 v27.25,59.76 | v30.8,59.76 30.8,59.88 31.87,60.95 31.87,69.07 33.34,70.53 45.13,70.53 46.55,71.95 v46.55,72.46
  Bottom 0.152: v89.79,55 v86.34,55 | v101,60.21 v101,63.66 | v95,44.11 v95,40.67 | v60.21,95 v63.66,95 | v49,89.79 v49,86.34 | v55,105.89 v55,109.33 | v43.92,79.35 43.92,77.96 44.3,77.58 44.77,77.58 46.55,75.8 v46.55,72.46 47.03,71.98 76.27,71.98 80.36,76.07 92.88,76.07 94.79,74.15 94.79,71.07 94.81,71.06 96.45,69.41 100.9,69.41 101.4,68.92 103.1,68.92 103.62,69.43 104.13,69.43 104.69,69.99 105.22,69.99 v106.08,70.84 | v27.25,59.76 v30.8,59.76
A_OSCENIN  (via drill 0.3, 0.35)
  Top 0.152: PKG4.10 106.74,45.17 106.44,45.47 106.44,59.01 105.01,60.44 104.04,60.44 103.72,60.77 102.81,60.77 102.48,61.09 99.75,61.09 99.42,60.77 v99,60.77 99,60.74 98.7,60.44 91.01,60.44 89.56,58.99 89.56,57.92 89.23,57.6 89.23,56.81 88.91,56.48 88.91,53.75 89.23,53.42 v89.23,53 89.56,52.67 89.56,44.99 91.04,43.51 92.12,43.51 92.4,43.23 96.67,43.23 v97,43.56 | v86.34,53 85.74,53.61 85.74,54.21 85.46,54.49 85.46,55.09 85.18,55.37 85.18,55.98 84.9,56.26 84.9,58.59 84.66,58.83 PKG4.90 | v99,63.66 99.61,64.26 100.21,64.26 100.49,64.54 101.09,64.54 101.37,64.82 101.98,64.82 102.26,65.1 104.49,65.1 104.83,65.44 PKG4.50 104.83,70.83 v104.78,70.87 | PKG1.10 43.26,104.83 43.56,104.53 43.56,90.99 44.99,89.56 45.96,89.56 46.28,89.23 47.19,89.23 47.52,88.91 50.25,88.91 50.58,89.23 v51,89.23 51,89.26 51.3,89.56 58.99,89.56 60.44,91.01 60.44,92.08 60.77,92.4 60.77,93.19 61.09,93.52 61.09,96.25 60.77,96.58 v60.77,97 60.44,97.33 60.44,105.01 58.96,106.49 57.88,106.49 57.6,106.77 53.33,106.77 v53,106.44 | v63.66,97 64.26,96.39 64.26,95.79 64.54,95.51 64.54,94.91 64.82,94.63 64.82,94.02 65.1,93.74 65.1,91.41 65.34,91.17 PKG1.90 | v51,86.34 50.39,85.74 49.79,85.74 49.51,85.46 48.91,85.46 48.63,85.18 48.02,85.18 47.74,84.9 45.51,84.9 45.17,84.56 PKG1.50 45.17,79.4 v45.22,79.35 | PKG1.130 58.83,111.05 58.55,110.77 56.26,110.77 55.98,110.5 55.52,110.5 55.24,110.22 54.31,110.22 v54.05,110.47 | v94.43,39.05 91.65,39.05 91.17,38.58 PKG4.130 | CN8.A13 6.25,64.82 16.56,64.82 CN4.A13 17.85,66.34 18.92,67.41 23.99,67.41 24.81,66.59 24.81,64.2 25.43,63.58 25.43,59.25 26.96,57.73 v27.25,57.73
  Top 0.152: v30.8,57.73 30.8,57.85 32.43,59.48 32.43,68.84 33.57,69.98 45.59,69.98 48.58,72.97 v48.58,73.48
  Bottom 0.152: v89.23,53 v86.34,53 | v99,60.77 v99,63.66 | v60.77,97 v63.66,97 | v51,89.23 v51,86.34 | v45.22,79.35 45.16,79.29 45.16,77.98 48.58,74.55 v48.58,73.48 49.52,72.54 76.04,72.54 80.12,76.63 93.11,76.63 95.35,74.39 95.35,71.3 96.69,69.97 101.14,69.97 101.63,69.47 102.87,69.47 103.39,69.99 103.9,69.99 v104.78,70.87 | v97,43.56 96.6,43.16 96.6,40.92 96.61,40.92 96.61,40.42 96.25,40.06 94.78,40.06 94.43,39.71 v94.43,39.05 | v53,106.44 53,110.12 53.35,110.47 v54.05,110.47 | v27.25,57.73 v30.8,57.73
A_OSCIN  (via drill 0.3, 0.35)
  Top 0.152: PKG4.7 105.86,43.23 105.61,43.48 105.61,58.66 104.66,59.61 103.7,59.61 103.37,59.93 v102,59.93 101.89,59.93 101.57,59.61 91.35,59.61 90.39,58.65 90.39,57.58 90.07,57.25 v90.07,56 90.39,55.67 90.39,45.34 91.34,44.39 92.42,44.39 92.75,44.07 93.67,44.07 v94,44.39 | v86.34,56 85.74,56.61 85.74,60.51 85.47,60.77 PKG4.87 | v102,63.66 102.61,64.26 106.36,64.26 106.78,64.67 PKG4.47 106.78,71.72 v106.68,71.82 | v94,40.67 93.39,40.06 89.56,40.06 89.22,39.73 PKG4.127 | PKG1.7 44.14,106.78 44.39,106.52 44.39,91.34 45.34,90.39 46.3,90.39 46.63,90.07 v48,90.07 48.11,90.07 48.43,90.39 58.65,90.39 59.61,91.35 59.61,92.42 59.93,92.75 v59.93,94 59.61,94.33 59.61,104.66 58.66,105.61 57.58,105.61 57.25,105.93 56.33,105.93 v56,105.61 | v63.66,94 64.26,93.39 64.26,89.49 64.53,89.22 PKG1.87 | v48,86.34 47.39,85.74 43.64,85.74 43.23,85.33 PKG1.47 43.23,78.27 v43.31,78.18 | v56,109.33 56.61,109.94 60.44,109.94 60.77,110.28 PKG1.127 | CN4.C15 22.99,71.25 25.86,71.25 26.4,70.71 26.4,67.73 25.65,66.99 25.65,64.55 26.27,63.93 26.27,61.28 26.78,60.78 v27.25,60.78 | v30.8,60.78 30.8,60.9 31.59,61.69 31.59,69.18 33.22,70.81 44.78,70.81 45.54,71.57 v45.54,71.95
  Route15 0.152: CN4.C15 21.64,72.48 11.33,72.48 CN8.C15
  Bottom 0.152: v90.07,56 v86.34,56 | v102,59.93 v102,63.66 | v94,44.39 v94,40.67 | v59.93,94 v63.66,94 | v48,90.07 v48,86.34 | v56,105.61 v56,109.33 | v43.31,78.18 43.31,78.12 44.13,77.3 44.65,77.3 45.54,76.42 v45.54,71.95 45.79,71.7 76.38,71.7 80.47,75.79 92.76,75.79 94.51,74.04 94.51,74 94.51,73.99 94.51,70.95 96.34,69.13 100.79,69.13 101.28,68.64 103.22,68.64 103.73,69.15 104.25,69.15 104.8,69.71 105.34,69.71 105.87,70.24 106.33,70.24 106.69,70.59 106.69,71.09 106.68,71.1 v106.68,71.82 | v27.25,60.78 v30.8,60.78
A_SHIFTCLKIN  (via drill 0.3)
  Top 0.152: PKG4.19 108.53,51.02 108.12,51.43 108.12,59.71 105.71,62.12 104.74,62.12 104.41,62.45 103.51,62.45 103.18,62.77 93.76,62.77 93.43,62.45 v93,62.45 92.67,62.12 90.31,62.12 87.88,59.69 87.88,58.62 87.55,58.29 87.55,57.5 87.23,57.18 87.23,47.73 87.55,47.41 v87.55,47 87.88,46.67 87.88,44.29 90.34,41.83 91.43,41.83 91.71,41.55 102.67,41.55 v103,41.88 | v86.34,47 85.74,47.61 85.74,48.21 85.46,48.49 85.46,49.09 85.18,49.37 85.18,49.98 84.9,50.26 84.9,50.86 84.62,51.14 84.62,51.75 84.34,52.03 84.34,52.63 84,52.98 PKG4.99 | v93,63.66 93.61,64.26 94.22,64.26 94.5,64.54 95.09,64.54 95.37,64.82 95.98,64.82 96.26,65.1 96.86,65.1 97.14,65.38 97.75,65.38 98.03,65.66 98.63,65.66 98.97,66 PKG4.59 98.97,71.76 v98.49,72.25 | v63.66,103 64.26,102.39 64.26,101.79 64.54,101.51 64.54,100.91 64.82,100.63 64.82,100.02 65.1,99.74 65.1,99.14 65.38,98.86 65.38,98.25 65.66,97.97 65.66,97.37 66,97.03 PKG1.99 | v57,86.34 56.39,85.74 55.78,85.74 55.5,85.46 54.91,85.46 54.63,85.18 54.02,85.18 53.74,84.9 53.14,84.9 52.86,84.62 52.25,84.62 51.97,84.34 51.37,84.34 51.02,84 PKG1.59 51.02,78.07 v50.71,77.75 | v47,108.12 47.33,108.45 58.29,108.45 58.57,108.17 59.66,108.17 62.12,105.71 62.12,103.33 v62.45,103 62.45,102.59 62.77,102.27 62.77,92.82 62.45,92.5 62.45,91.71 62.12,91.38 62.12,90.31 59.69,87.88 57.33,87.88 v57,87.55 56.57,87.55 56.24,87.23 46.82,87.23 46.49,87.55 45.59,87.55 45.26,87.88 44.29,87.88 41.88,90.29 41.88,98.57 41.48,98.97 PKG1.19 32.19,98.97 v31.75,99.41 | v26.26,99.53 26.26,99.32 25.65,98.71 25.65,98.17 26.3,97.52 26.3,96.33 26.68,95.95 26.68,94.14 26.02,93.48 26.02,90.4 26.4,90.03 26.4,81.16 25.27,80.04 18.82,80.04 17.85,79.07 CN4.A18 16.55,77.51 6.26,77.51 CN8.A18
  Top 0.152: v103,40.67 103,39.63 102.81,39.44 101.13,39.44 100.01,38.32 98,38.32 97.03,37.34 PKG4.139 | PKG1.139 52.98,112.19 52.8,112.01 52.47,112.01 52.14,111.68 50.11,111.68 48.95,110.52 47.34,110.52 47.06,110.24 47.06,109.39 v47,109.33
  Bottom 0.152: v87.55,47 v86.34,47 | v93,62.45 v93,63.66 | v103,41.88 v103,40.67 | v62.45,103 v63.66,103 | v57,87.55 v57,86.34 | v47,108.12 v47,109.33 | v50.71,77.75 51.37,77.09 51.37,75.88 53.04,74.21 69.53,74.21 73.62,78.3 93.8,78.3 97.03,75.08 97.03,72 97.38,71.64 97.88,71.64 98.23,72 98.23,72.23 98.25,72.25 v98.49,72.25 | v31.75,99.41 26.38,99.41 v26.26,99.53
A_SHIFTIN  (via drill 0.3)
  Top 0.152: PKG4.12 107.31,46.48 107,46.78 107,59.24 105.24,61 104.28,61 103.95,61.33 103.04,61.33 102.71,61.65 97.75,61.65 97.42,61.33 v97,61.33 96.67,61 90.78,61 89,59.22 89,58.16 88.67,57.83 88.67,57.04 88.35,56.71 88.35,51.75 88.67,51.42 v88.67,51 89,50.67 89,44.76 90.81,42.95 91.89,42.95 92.17,42.67 98.67,42.67 v99,43 | v86.34,51 85.74,51.61 85.74,52.21 85.46,52.49 85.46,53.09 85.18,53.37 85.18,53.98 84.9,54.26 84.9,54.86 84.62,55.14 84.62,55.75 84.34,56.03 84.34,57.21 84.03,57.52 PKG4.92 | v97,63.66 97.61,64.26 98.21,64.26 98.49,64.54 99.09,64.54 99.37,64.82 99.98,64.82 100.26,65.1 100.86,65.1 101.14,65.38 101.75,65.38 102.03,65.66 103.19,65.66 103.53,66 PKG4.52 103.53,70.83 v103.48,70.88 | v63.66,99 64.26,98.39 64.26,97.79 64.54,97.51 64.54,96.91 64.82,96.63 64.82,96.02 65.1,95.74 65.1,95.14 65.38,94.86 65.38,94.25 65.66,93.97 65.66,92.79 65.97,92.47 PKG1.92 | v53,86.34 52.39,85.74 51.79,85.74 51.51,85.46 50.91,85.46 50.63,85.18 50.02,85.18 49.74,84.9 49.14,84.9 48.86,84.62 48.25,84.62 47.97,84.34 46.81,84.34 46.48,84 PKG1.52 46.48,79.4 v46.52,79.35 | v51,107 51.33,107.33 57.83,107.33 58.11,107.05 59.2,107.05 61,105.24 61,99.33 v61.33,99 61.33,98.58 61.65,98.25 61.65,93.29 61.33,92.96 61.33,92.17 61,91.84 61,90.78 59.22,89 53.33,89 v53,88.67 52.58,88.67 52.25,88.35 47.29,88.35 46.96,88.67 46.05,88.67 45.73,89 44.76,89 43,90.76 43,103.22 42.69,103.53 PKG1.12 33.3,103.53 33.01,103.82 33.01,104.66 32.76,104.91 v32.18,104.91 | v26.63,105.35 26.63,105.16 25.75,104.27 25.75,101.73 25.09,101.08 25.09,100.62 24.53,100.06 24.53,97.7 25.19,97.05 25.19,95.86 25.56,95.49 25.56,94.6 24.91,93.95 24.91,89.94 25.28,89.57 25.28,85.62 24.84,85.18 18.98,85.18 17.85,84.05 CN4.A20 16.59,82.63 6.22,82.63 CN8.A20
  Top 0.152: v99,40.67 99,39.68 98.75,39.43 97.54,39.43 96.69,38.59 95.67,38.59 95.25,38.16 92.91,38.16 92.47,37.73 PKG4.132 | v51,109.33 51,110.31 51.26,110.57 52.6,110.57 52.93,110.9 53.27,110.9 53.64,111.27 54.39,111.27 54.8,111.68 56.21,111.68 56.56,112.03 57.25,112.03 57.52,112.31 PKG1.132
  Bottom 0.152: v88.67,51 v86.34,51 | v97,61.33 v97,63.66 | v99,43 v99,40.67 | v61.33,99 v63.66,99 | v53,88.67 v53,86.34 | v51,107 v51,109.33 | v46.52,79.35 46.41,79.25 46.41,77.88 46.72,77.58 46.97,77.58 51.45,73.09 69.99,73.09 74.08,77.18 93.34,77.18 95.91,74.62 95.91,71.53 96.92,70.53 101.37,70.53 101.86,70.03 102.64,70.03 v103.48,70.88 | v32.18,104.91 27.07,104.91 v26.63,105.35
A_SIN  (via drill 0.3, 0.35)
  Top 0.152: PKG4.6 105.59,42.58 105.33,42.84 105.33,58.55 104.55,59.33 v103,59.33 91.47,59.33 90.67,58.53 v90.67,57 90.67,45.45 91.45,44.67 v93,44.67 | v86.34,57 86.34,61.11 86.03,61.42 PKG4.86 | v103,63.66 106.97,63.66 107.42,64.11 PKG4.46 107.42,70.79 v107.38,70.83 | v93,40.67 88.88,40.67 88.58,40.37 PKG4.126 | PKG1.6 44.41,107.42 44.67,107.16 44.67,91.45 45.45,90.67 v47,90.67 58.53,90.67 59.33,91.47 v59.33,93 59.33,104.55 58.55,105.33 v57,105.33 | v63.66,93 63.66,88.89 63.98,88.58 PKG1.86 | v47,86.34 43.03,86.34 42.58,85.89 PKG1.46 42.58,79.4 v42.62,79.35 | v57,109.33 61.12,109.33 61.42,109.63 PKG1.126 | CN8.A15 6.24,69.91 16.57,69.91 CN4.A15 17.85,71.33 18.95,72.43 25.76,72.43 26.68,71.51 26.68,67.62 25.93,66.87 25.93,64.66 26.58,64.01 26.58,62.3 27.09,61.79 v27.25,61.79 | v30.8,61.79 31.31,62.3 31.31,69.41 33.34,71.44 v44.52,71.44
  Bottom 0.152: v90.67,57 v86.34,57 | v103,59.33 v103,63.66 | v93,44.67 v93,40.67 | v59.33,93 v63.66,93 | v47,90.67 v47,86.34 | v57,105.33 v57,109.33 | v42.62,79.35 42.62,78.02 43.06,77.58 43.46,77.58 44.52,76.52 v44.52,71.44 44.64,71.32 45.8,71.32 45.89,71.42 76.5,71.42 80.59,75.51 92.6,75.51 94.23,73.88 94.23,70.84 96.22,68.85 100.67,68.85 101.16,68.36 103.33,68.36 103.85,68.87 104.36,68.87 104.92,69.43 105.45,69.43 105.99,69.96 106.51,69.96 v107.38,70.83 | v27.25,61.79 v30.8,61.79
A_SRSTIN  (via drill 0.3, 0.35)
  Top 0.152: PKG4.9 106.41,44.52 106.16,44.78 106.16,58.9 104.9,60.16 103.93,60.16 103.6,60.49 102.69,60.49 102.37,60.82 100.75,60.82 100.42,60.49 v100,60.49 99.67,60.16 91.12,60.16 89.84,58.88 89.84,57.81 89.51,57.48 89.51,56.69 89.18,56.37 89.18,54.75 89.51,54.42 v89.51,54 89.84,53.67 89.84,45.1 91.15,43.79 92.24,43.79 92.52,43.51 95.67,43.51 v96,43.84 | v86.34,54 85.74,54.61 85.74,55.21 85.46,55.49 85.46,56.09 85.18,56.37 85.18,59.24 84.94,59.48 PKG4.89 | v100,63.66 100.61,64.26 101.21,64.26 101.49,64.54 102.09,64.54 102.37,64.82 105.11,64.82 105.47,65.19 PKG4.49 105.47,71.73 v105.39,71.82 | v96,40.67 95.86,40.67 95.25,40.06 94.65,40.06 94.37,39.78 93.91,39.78 93.63,39.51 90.73,39.51 90.53,39.3 PKG4.129 | PKG1.9 43.59,105.47 43.84,105.22 43.84,91.1 45.1,89.84 46.07,89.84 46.4,89.51 47.31,89.51 47.63,89.18 49.25,89.18 49.58,89.51 v50,89.51 50.33,89.84 58.88,89.84 60.16,91.12 60.16,92.19 60.49,92.52 60.49,93.31 60.82,93.63 60.82,95.25 60.49,95.58 v60.49,96 60.16,96.33 60.16,104.9 58.85,106.21 57.76,106.21 57.48,106.49 54.33,106.49 v54,106.16 | v63.66,96 64.26,95.39 64.26,94.79 64.54,94.51 64.54,93.91 64.82,93.63 64.82,90.76 65.06,90.53 PKG1.89 | v50,86.34 49.39,85.74 48.79,85.74 48.51,85.46 47.91,85.46 47.63,85.18 44.89,85.18 44.52,84.81 PKG1.49 44.52,78.22 v44.56,78.18 | v54,109.33 54.14,109.33 54.75,109.94 55.35,109.94 55.63,110.22 56.09,110.22 56.37,110.5 59.27,110.5 59.48,110.7 PKG1.129 | CN4.C14 22.97,68.61 24.41,68.61 25.09,67.93 25.09,64.32 25.71,63.7 25.71,59.88 26.85,58.74 v27.25,58.74 | v30.8,58.74 30.8,58.87 32.15,60.22 32.15,68.95 33.45,70.25 45.36,70.25 47.57,72.46 v47.57,72.97
  Route15 0.152: CN4.C14 21.64,69.94 11.33,69.94 CN8.C14
  Bottom 0.152: v89.51,54 v86.34,54 | v100,60.49 v100,63.66 | v96,43.84 v96,40.67 | v60.49,96 v63.66,96 | v50,89.51 v50,86.34 | v54,106.16 v54,109.33 | v44.56,78.18 47.57,75.17 v47.57,72.97 48.28,72.26 76.15,72.26 80.24,76.35 92.99,76.35 95.07,74.27 95.07,71.19 96.57,69.69 101.02,69.69 101.51,69.19 102.98,69.19 103.5,69.71 104.02,69.71 104.57,70.27 105.09,70.27 105.39,70.57 v105.39,71.82 | v27.25,58.74 v30.8,58.74
A_STVCLKIN  (via drill 0.3)
  Top 0.152: PKG4.20 108.85,51.67 108.4,52.13 108.4,59.82 105.82,62.4 104.85,62.4 104.53,62.73 103.63,62.73 103.3,63.05 92.42,63.05 92.39,63.08 | 92.39,63.08 92.39,62.7 92.1,62.4 90.2,62.4 87.6,59.8 87.6,58.73 87.28,58.41 87.28,57.62 86.95,57.29 86.95,46.43 86.98,46.39 | 92.39,63.08 92.39,63.95 92.98,64.54 94.1,64.54 94.38,64.82 94.98,64.82 95.26,65.1 95.86,65.1 96.14,65.38 96.75,65.38 97.03,65.66 97.63,65.66 97.91,65.94 98.17,65.94 98.33,66.09 PKG4.60 98.33,71.55 v97.63,72.25 | PKG4.100 83.91,52.33 84.06,52.17 84.06,51.91 84.34,51.63 84.34,51.03 84.62,50.75 84.62,50.14 84.9,49.86 84.9,49.26 85.18,48.98 85.18,48.37 85.46,48.09 85.46,47.03 86.09,46.39 86.98,46.39 | 86.98,46.39 87.22,46.39 87.6,46.02 87.6,44.18 90.23,41.55 91.31,41.55 91.59,41.27 103.25,41.27 103.61,40.92 103.61,39.53 103.23,39.16 101.24,39.16 100.12,38.04 98.12,38.04 97.71,37.63 97.71,35.88 PKG4.140 | 57.61,86.92 57.61,87.3 57.9,87.6 59.8,87.6 62.4,90.2 62.4,91.27 62.73,91.59 62.73,92.38 63.05,92.71 63.05,103.57 63.02,103.61 | 57.61,86.92 57.61,86.05 57.02,85.46 55.9,85.46 55.62,85.18 55.02,85.18 54.74,84.9 54.14,84.9 53.86,84.62 53.25,84.62 52.97,84.34 52.37,84.34 52.09,84.06 51.83,84.06 51.67,83.91 PKG1.60 v51.67,77.76 v51.68,77.75 | 57.61,86.92 57.58,86.95 46.7,86.95 46.37,87.28 45.47,87.28 45.15,87.6 44.18,87.6 41.6,90.18 41.6,97.87 41.15,98.33 PKG1.20 31.8,98.33 v31.75,98.37 | PKG1.100 66.09,97.67 65.94,97.83 65.94,98.09 65.66,98.37 65.66,98.97 65.38,99.25 65.38,99.86 65.1,100.14 65.1,100.74 64.82,101.02 64.82,101.63 64.54,101.91 64.54,102.97 63.91,103.61 63.02,103.61
  Top 0.152: 63.02,103.61 62.77,103.61 62.4,103.98 62.4,105.82 59.77,108.45 58.69,108.45 58.41,108.72 46.75,108.72 46.39,109.08 46.39,109.58 46.78,109.97 46.78,110.36 47.22,110.8 48.83,110.8 49.99,111.96 52.02,111.96 52.33,112.27 PKG1.140 | v26.26,98.46 26.58,98.13 26.58,96.44 26.96,96.07 26.96,94.02 26.3,93.37 26.3,90.52 26.68,90.15 26.68,80.61 24.88,78.81 CN4.C18
  Route15 0.152: CN4.C18 21.66,80.08 11.31,80.08 CN8.C18
  Bottom 0.152: v51.68,77.75 51.65,77.72 51.65,76 53.16,74.49 69.41,74.49 73.5,78.58 93.92,78.58 97.3,75.19 97.3,72.57 v97.63,72.25 | v26.26,98.46 31.67,98.46 v31.75,98.37
A_STVSELIN  (via drill 0.3)
  Top 0.152: PKG4.13 107.63,47.12 107.28,47.48 107.28,59.36 105.36,61.28 104.39,61.28 104.06,61.61 103.16,61.61 102.83,61.93 96.75,61.93 96.42,61.61 v96,61.61 95.67,61.28 90.66,61.28 88.72,59.34 88.72,58.27 88.39,57.95 88.39,57.16 88.07,56.83 88.07,50.75 88.39,50.42 v88.39,50 88.72,49.67 88.72,44.64 90.69,42.67 91.78,42.67 92.06,42.39 99.67,42.39 v100,42.72 | v86.34,50 85.74,50.61 85.74,51.21 85.46,51.49 85.46,52.09 85.18,52.37 85.18,52.98 84.9,53.26 84.9,53.86 84.62,54.14 84.62,54.75 84.34,55.03 84.34,55.63 84.06,55.91 84.06,56.61 83.81,56.86 81.86,56.86 PKG4.93 | v96,63.66 96.61,64.26 97.21,64.26 97.49,64.54 98.09,64.54 98.37,64.82 98.98,64.82 99.26,65.1 99.86,65.1 100.14,65.38 100.75,65.38 101.03,65.66 101.63,65.66 101.91,65.94 102.55,65.94 102.88,66.27 PKG4.53 102.88,71.75 v102.81,71.82 | v63.66,100 64.26,99.39 64.26,98.79 64.54,98.51 64.54,97.91 64.82,97.63 64.82,97.02 65.1,96.74 65.1,96.14 65.38,95.86 65.38,95.25 65.66,94.97 65.66,94.37 65.94,94.09 65.94,93.39 66.19,93.14 68.14,93.14 PKG1.93 | v54,86.34 53.39,85.74 52.79,85.74 52.51,85.46 51.91,85.46 51.63,85.18 51.02,85.18 50.74,84.9 50.14,84.9 49.86,84.62 49.25,84.62 48.97,84.34 48.37,84.34 48.09,84.06 47.45,84.06 47.12,83.73 PKG1.53 47.12,78.29 v47.02,78.18 | v50,107.28 50.33,107.61 57.95,107.61 58.22,107.33 59.31,107.33 61.28,105.36 61.28,100.33 v61.61,100 61.61,99.58 61.93,99.25 61.93,93.17 61.61,92.84 61.61,92.06 61.28,91.73 61.28,90.66 59.34,88.72 54.33,88.72 v54,88.39 53.58,88.39 53.25,88.07 47.17,88.07 46.84,88.39 45.94,88.39 45.61,88.72 44.64,88.72 42.72,90.64 42.72,102.52 42.37,102.88 PKG1.13 33.06,102.88 32.18,103.76 v32.18,103.88
  Top 0.152: v26.63,104.3 26.02,103.69 26.02,101.62 25.37,100.97 25.37,100.51 24.81,99.95 24.81,97.82 25.47,97.17 25.47,95.98 25.84,95.61 25.84,94.48 25.19,93.83 25.19,90.24 25.19,90.09 25.19,90.06 25.56,89.69 25.56,84.34 25.04,83.82 23,83.82 CN4.C20 | v100,40.67 100,39.49 99.66,39.16 97.65,39.16 96.81,38.31 95.79,38.31 95.36,37.88 93.52,37.88 93.12,37.49 PKG4.133 | v50,109.33 50,110.39 50.45,110.84 52.49,110.84 52.81,111.17 53.15,111.17 53.53,111.55 54.27,111.55 54.68,111.96 56.1,111.96 56.88,112.74 PKG1.133
  Route15 0.152: CN4.C20 21.68,85.14 11.29,85.14 CN8.C20
  Bottom 0.152: v88.39,50 v86.34,50 | v96,61.61 v96,63.66 | v100,42.72 v100,40.67 | v61.61,100 v63.66,100 | v54,88.39 v54,86.34 | v50,107.28 v50,109.33 | v47.02,78.18 47.02,77.92 51.56,73.37 69.88,73.37 73.96,77.46 93.45,77.46 96.19,74.73 96.19,71.65 97.03,70.8 101.48,70.8 101.97,70.31 102.48,70.31 102.86,70.69 102.86,71.77 v102.81,71.82 | v32.18,103.88 27.05,103.88 v26.63,104.3
A_STVSIN  (via drill 0.3)
  Top 0.152: PKG4.14 108.08,47.77 107.56,48.29 107.56,59.48 105.47,61.56 104.51,61.56 104.18,61.89 103.27,61.89 102.94,62.21 95.75,62.21 95.42,61.89 v95,61.89 94.67,61.56 90.54,61.56 88.44,59.46 88.44,58.39 88.11,58.06 88.11,57.27 87.79,56.95 87.79,49.75 88.11,49.42 v88.11,49 88.44,48.67 88.44,44.52 90.57,42.39 91.66,42.39 91.94,42.11 100.67,42.11 v101,42.44 | v86.34,49 85.74,49.61 85.74,50.21 85.46,50.49 85.46,51.09 85.18,51.37 85.18,51.98 84.9,52.26 84.9,52.86 84.62,53.14 84.62,53.75 84.34,54.03 84.34,54.63 84.06,54.91 84.06,55.52 83.78,55.8 83.78,56.08 83.64,56.23 PKG4.94 | v95,63.66 95.61,64.26 96.21,64.26 96.49,64.54 97.09,64.54 97.37,64.82 97.98,64.82 98.26,65.1 98.86,65.1 99.14,65.38 99.75,65.38 100.03,65.66 100.63,65.66 100.91,65.94 101.52,65.94 101.8,66.22 101.96,66.22 102.22,66.48 PKG4.54 102.22,70.96 v102.23,70.92 | v63.66,101 64.26,100.39 64.26,99.79 64.54,99.51 64.54,98.91 64.82,98.63 64.82,98.02 65.1,97.74 65.1,97.14 65.38,96.86 65.38,96.25 65.66,95.97 65.66,95.37 65.94,95.09 65.94,94.48 66.22,94.2 66.22,93.92 66.36,93.78 PKG1.94 | v55,86.34 54.39,85.74 53.79,85.74 53.51,85.46 52.91,85.46 52.63,85.18 52.02,85.18 51.74,84.9 51.14,84.9 50.86,84.62 50.25,84.62 49.97,84.34 49.37,84.34 49.09,84.06 48.48,84.06 48.2,83.78 48.04,83.78 47.77,83.52 PKG1.54 v47.77,79.35 v47.78,79.35 | v49,107.56 49.33,107.89 58.06,107.89 58.34,107.61 59.43,107.61 61.56,105.47 61.56,101.33 v61.89,101 61.89,100.58 62.21,100.25 62.21,93.06 61.89,92.73 61.89,91.94 61.56,91.61 61.56,90.54 59.46,88.44 55.33,88.44 v55,88.11 54.58,88.11 54.25,87.79 47.05,87.79 46.73,88.11 45.82,88.11 45.49,88.44 44.52,88.44 42.44,90.53 42.44,101.71 41.92,102.22 PKG1.14 32.82,102.22 v32.18,102.86
  Top 0.152: v26.63,103.27 26.3,102.95 26.3,101.5 25.65,100.85 25.65,100.39 25.09,99.83 25.09,97.94 25.75,97.28 25.75,96.09 26.12,95.72 26.12,94.37 25.47,93.72 25.47,90.17 25.84,89.8 25.84,82.94 25.43,82.53 19.01,82.53 17.85,81.37 CN4.A19 16.6,80.1 6.21,80.1 CN8.A19 | v101,40.67 101,40.1 99.78,38.88 97.77,38.88 96.92,38.03 95.9,38.03 95.48,37.6 94.03,37.6 93.78,37.34 PKG4.134 | v49,109.33 49,109.79 50.34,111.12 52.37,111.12 52.7,111.45 53.03,111.45 53.41,111.83 54.16,111.83 54.56,112.24 55.98,112.24 56.23,112.48 PKG1.134
  Bottom 0.152: v88.11,49 v86.34,49 | v95,61.89 v95,63.66 | v101,42.44 v101,40.67 | v61.89,101 v63.66,101 | v55,88.11 v55,86.34 | v49,107.56 v49,109.33 | v102.23,70.92 102.06,71.08 97.15,71.08 96.47,71.77 96.47,74.85 93.57,77.74 73.85,77.74 69.76,73.65 51.68,73.65 47.62,77.71 47.62,79.2 v47.78,79.35 | v26.63,103.27 31.77,103.27 v32.18,102.86
B1/CLK_OUT  (via drill 0.35)
  Top 0.152: CN1.C17 v73.73,24.84 | JP1.2 56.96,68.66 57.3,69 65.7,69 68.8,65.91 v68.8,64.4 | v73.73,27.38 72.74,28.37 72.74,35.96 69.84,38.86 69.84,44.95 70.63,45.74 70.63,46.26 69.56,47.33 69.56,58.96 v70,59.4
  Route15 0.152: CN5.C17 72.46,11.31 72.46,21.66 CN1.C17
  Bottom 0.152: v73.73,24.84 v73.73,27.38 | v70,59.4 70.83,60.23 70.83,62.37 v68.8,64.4
B1/S_OUT  (via drill 0.35)
  Top 0.152: CN3.C15 71.19,116.51 74.25,113.45 74.25,108.54 74.9,107.89 74.9,86.87 75.18,86.59 75.18,82.8 74.91,82.53 74.91,65.81 71.2,62.1 v70.2,62.1
  Route15 0.152: CN7.C15 72.46,138.69 72.46,128.34 CN3.C15
  Bottom 0.152: v70.2,62.1 69,62.1 68.8,62.1 66.56,62.1 JP2.2
B2/CLK_OUT  (via drill 0.35)
  Top 0.152: CN5.A17 75,6.23 75,16.58 CN1.A17 72.46,19.12 v72.46,24.84 | v72.46,27.38 72.46,35.84 69.56,38.74 69.56,45.56 v70,46
  Bottom 0.152: v72.46,24.84 v72.46,27.38 | v70,46 70,46.6 69.5,47.1 66.56,47.1 JP3.2
B2/S_OUT  (via drill 0.35)
  Top 0.152: CN3.C16 v73.73,115.64 | v75,111.83 75,108.19 75.18,108.01 75.18,86.99 75.46,86.71 75.46,82.69 75.19,82.42 75.19,65.7 69.28,59.79 69.28,38.38 65.19,34.3 v62.5,34.3
  Route15 0.152: CN7.C16 75,138.69 75,128.34 CN3.C16
  Bottom 0.152: v73.73,115.64 75,114.37 v75,111.83 | v62.5,34.3 62.1,34.7 62.1,37.44 JP4.2
B3/CLK_OUT  (via drill 0.35)
  Top 0.152: CN1.C18 v71.19,24.84 | v71.19,27.38 71.19,32.45 70.28,33.37 59.44,33.37 58.45,34.36 48.26,34.36 47.9,34 v47.3,34
  Route15 0.152: CN5.C18 69.92,11.31 69.92,21.66 CN1.C18
  Bottom 0.152: v71.19,24.84 v71.19,27.38 | JP5.2 47.04,34.26 v47.3,34
B3/S_OUT  (via drill 0.35)
  Top 0.152: CN3.C13 66.11,124.19 63.57,121.65 56.63,121.65 55.98,122.3 55.24,122.3 54.31,121.37 48.43,121.37 47.22,122.58 45.17,122.58 44.52,121.93 35.84,121.93 28.07,114.16 28.07,112.36 26.86,111.15 26.86,108.92 27.52,108.27 27.52,102.79 26.86,102.14 26.86,101.55 27.79,100.62 27.79,99.68 27.14,99.03 27.14,96.67 27.52,96.3 27.52,93.79 26.86,93.14 26.86,90.75 27.24,90.38 27.24,78.68 26.53,77.98 26.53,73.51 26.74,73.3 v26.74,72.46 | v34,68.5 34,66 34.44,65.56 34.44,56.63 33.37,55.56 33.37,55.04 34.16,54.25 34.16,45.85 33.39,45.08 33.39,44.32 33.5,44.21 v33.5,43.5
  Route2 0.152: v26.74,72.46 27.2,72 31,72 34,69 v34,68.5
  Route15 0.152: CN7.C13 67.38,138.69 67.38,128.34 CN3.C13
  Bottom 0.152: v33.5,43.5 35.04,41.96 JP6.2
B4/CLK_OUT  (via drill 0.35)
  Top 0.152: CN5.A18 72.46,6.23 72.46,16.58 CN1.A18 69.92,19.12 v69.92,24.84 | v69.92,27.38 69.92,32.45 69.28,33.09 59.32,33.09 58.36,34.05 48.35,34.05 47.66,33.37 46.93,33.37 45.86,34.44 38.77,34.44 34.44,38.77 34.44,43.67 33.67,44.44 33.67,44.96 34.44,45.73 34.44,54.86 v34,55.3
  Bottom 0.152: v69.92,24.84 v69.92,27.38 | v34,55.3 34,56.7 34.15,56.85 34.2,56.9 34.26,56.96 JP7.2
B4/S_OUT  (via drill 0.35)
  Top 0.152: v26.1,78.81 26.1,79.44 26.96,80.3 26.96,90.26 26.58,90.64 26.58,93.25 27.24,93.9 27.24,96.19 26.86,96.56 26.86,101.15 26.58,101.43 26.58,102.26 27.24,102.91 27.24,108.15 26.58,108.8 26.58,111.27 27.79,112.48 27.79,114.28 35.72,122.21 44.41,122.21 45.06,122.86 47.33,122.86 48.54,121.65 54.2,121.65 55.13,122.58 56.09,122.58 56.74,121.93 63.45,121.93 64.84,123.31 64.84,130.88 CN3.A13 67.38,133.42 67.38,143.77 CN7.A13
  Bottom 0.152: v26.1,78.81 26.74,78.17 29.91,78.17 37.07,71.02 37.07,68.44 37.49,68.02 41.34,68.02 41.96,67.4 JP8.2
B5/CLK_OUT  (via drill 0.35)
  Top 0.152: CN1.C14 v81.35,24.84 | v81.35,27.38 82.62,28.65 85.6,28.65 86.05,29.1 86.84,29.1 87.46,29.72 102.18,29.72 102.83,29.07 103.57,29.07 103.97,29.47 113.59,29.47 120.53,36.41 120.53,38.3 121.18,38.95 121.18,39.69 120.25,40.62 120.25,52.09 120.81,52.65 120.81,55.88 121.46,56.53 121.46,58.13 120.81,58.78 120.81,67.69 119.69,68.8 119.69,75.95 116.28,79.37 105.44,79.37 104.44,80.36 94.26,80.36 93.9,80 v93.3,80
  Route15 0.152: CN1.C14 80.08,21.66 80.08,11.31 CN5.C14
  Bottom 0.152: v81.35,24.84 v81.35,27.38 | v93.3,80 93.1,80.2 93.1,81.5 93.1,81.7 93.1,83.44 JP9.2
B5/S_OUT  (via drill 0.35)
  Top 0.152: CN7.A17 77.54,143.77 77.54,133.42 CN3.A17 75,130.88 75,113.5 75.91,112.58 75.91,91.87 v79.44,88.34
  Bottom 0.152: v79.44,88.34 79.82,87.96 JP10.2
B6/CLK_OUT  (via drill 0.35)
  Top 0.152: CN5.A14 82.62,6.23 82.62,16.58 CN1.A14 80.08,19.12 v80.08,24.84 | v80.08,27.38 81.63,28.92 85.48,28.92 85.94,29.38 86.72,29.38 87.34,30 102.3,30 102.95,29.35 103.45,29.35 103.86,29.75 113.47,29.75 120.25,36.53 120.25,38.42 120.9,39.07 120.9,39.57 119.97,40.5 119.97,52.21 120.53,52.77 120.53,56 121.18,56.65 121.18,58.01 120.53,58.66 120.53,67.57 119.41,68.69 119.41,75.84 116.16,79.09 105.32,79.09 104.36,80.06 94.35,80.06 93.66,79.37 92.93,79.37 91.86,80.44 84.77,80.44 80.44,84.77 80.44,89.27 79.67,90.04 79.67,90.96 80.44,91.73 80.44,100.86 v80,101.3
  Bottom 0.152: v80.08,24.84 v80.08,27.38 | v80,101.3 80,102.7 80.15,102.85 80.2,102.9 80.26,102.96 JP11.2
B6/S_OUT  (via drill 0.35)
  Top 0.152: v81.98,114.37 78.81,117.55 76.91,117.55 76.27,118.18 CN3.C17
  Route15 0.152: CN3.C17 77.54,128.34 77.54,138.69 CN7.C17
  Bottom 0.152: JP12.2 87.96,113.4 87.34,114.02 82.34,114.02 v81.98,114.37
B7/CLK_OUT  (via drill 0.35)
  Top 0.152: CN1.C13 v83.89,24.84 | v83.89,27.38 84.53,28.01 85.75,28.01 86.28,28.54 87.07,28.54 87.69,29.16 101.95,29.16 102.6,28.51 103.8,28.51 104.2,28.91 113.82,28.91 121.09,36.18 121.09,38.07 121.74,38.72 121.74,39.92 120.81,40.85 120.81,51.86 121.37,52.42 121.37,55.65 122.02,56.3 122.02,58.36 121.37,59.01 121.37,67.92 120.25,69.03 120.25,76.19 118.88,77.56 118.88,81.82 115.84,84.86 115.84,90.95 116.63,91.74 116.63,92.26 115.56,93.33 115.56,104.96 v116,105.4 | JP13.2 102.96,114.66 103.3,115 111.7,115 114.8,111.91 v114.8,111.03
  Route15 0.152: CN1.C13 82.62,21.66 82.62,11.31 CN5.C13
  Bottom 0.152: v83.89,24.84 v83.89,27.38 | v116,105.4 116.83,106.23 116.83,109 v114.8,111.03
B7/S_OUT  (via drill 0.35)
  Top 0.152: CN3.C18 78.81,122.62 85.88,115.56 111.94,115.56 116.2,111.3 v116.2,108.73
  Route15 0.152: CN3.C18 80.08,128.34 80.08,138.69 CN7.C18
  Bottom 0.152: v116.2,108.73 115.56,108.1 115,108.1 114.8,108.1 112.56,108.1 JP14.2
B8/CLK_OUT  (via drill 0.35)
  Top 0.152: CN5.A13 85.16,6.23 85.16,16.58 CN1.A13 82.62,19.12 v82.62,24.84 | v82.62,27.38 83.53,28.29 85.64,28.29 86.17,28.82 86.96,28.82 87.58,29.44 102.07,29.44 102.72,28.79 103.68,28.79 104.09,29.19 113.7,29.19 120.81,36.3 120.81,38.19 121.46,38.84 121.46,39.8 120.53,40.73 120.53,51.98 121.09,52.54 121.09,55.77 121.74,56.42 121.74,58.24 121.09,58.89 121.09,67.8 119.97,68.92 119.97,76.07 118.6,77.44 118.6,81.7 115.56,84.74 115.56,91.56 v116,92
  Bottom 0.152: v82.62,24.84 v82.62,27.38 | v116,92 116,92.6 115.5,93.1 114.5,93.1 114.3,93.1 112.56,93.1 JP15.2
B8/S_OUT  (via drill 0.35)
  Top 0.152: v108.5,80.3 111.19,80.3 115.28,84.38 115.28,98.17 114.69,98.76 v114.69,100.4 | v116.59,102.94 116.59,105.1 116.83,105.34 116.83,111.06 112.05,115.84 86.11,115.84 83.89,118.06 v83.89,120.72 | CN3.C20 v83.89,122.94
  Route15 0.152: CN7.C20 85.16,138.69 85.16,128.34 CN3.C20
  Bottom 0.152: v108.5,80.3 108.1,80.7 108.1,83.44 JP16.2 | v114.69,100.4 114.69,100.72 116.59,102.62 v116.59,102.94 | v83.89,120.72 v83.89,122.94
FR_CI  (via drill 0.3)
  Top 0.152: PKG4.111 78.34,45.17 77.98,44.81 77.98,43.17 78.69,42.47 78.69,40.23 82.99,35.93 v83.45,35.93 | PKG1.111 71.66,104.83 72.02,105.19 72.02,107.26 71.36,107.91 71.36,109.52 66.66,114.23 v66.26,114.23 | v66.26,120.3 65.93,120.62 64.2,120.62 64.11,120.53 48.08,120.53 47.15,121.46 46.56,121.46 45.91,120.81 36.3,120.81 29.19,113.7 29.19,111.9 28.26,110.97 28.26,110.42 28.91,109.77 28.91,99.22 28.26,98.56 28.26,97.14 28.63,96.76 28.63,93.33 27.98,92.67 27.98,91.25 28.35,90.87 28.35,77.75 v28.03,77.43 | v28.03,77.43 28.35,77.1 28.35,65.74 28.26,65.64 28.26,62.92 28.88,62.3 28.88,48.25 28.88,35.03 36.67,27.24 63.78,27.24 64.44,26.58 84.63,26.58 v84.66,26.61 | v28.03,77.43 | v25.65,77.43 18.91,77.43 17.85,76.37 CN4.A17 16.54,74.96 6.27,74.96 CN8.A17
  Bottom 0.152: v66.26,114.23 v66.26,120.29 v66.26,120.3 | v28.03,77.43 v25.65,77.43 | v84.66,26.61 84.66,28.54 83.45,29.75 v83.45,35.93
FR_SI  (via drill 0.3)
  Top 0.152: PKG4.3 117.6,40.62 v117.82,40.84 | PKG1.3 32.4,109.38 v32.18,109.16 | v27.75,109.29 28.07,108.96 28.07,99.56 27.42,98.91 27.42,96.79 27.79,96.42 27.79,93.67 27.14,93.02 27.14,90.9 27.52,90.53 27.52,78.56 26.86,77.91 26.86,74.04 v27.14,73.76 27.52,73.39 27.52,67.27 26.77,66.53 26.77,65.01 27.42,64.36 27.42,62.57 28.04,61.95 28.04,46.44 27.33,45.73 27.33,45.14 28,44.48 28,34.72 36.33,26.4 63.44,26.4 64.09,25.75 83.88,25.75 84.53,25.09 86.06,25.09 86.58,25.61 86.58,27.65 86.63,27.7 87.42,27.7 88.04,28.32 101.6,28.32 102.25,27.67 104.18,27.67 104.51,27.34 105.01,27.34 105.74,28.07 114.16,28.07 121.93,35.84 121.93,37.72 122.58,38.38 122.58,41 v122,41.58 | CN4.C16 22.95,73.75 v25.65,73.75
  Route15 0.152: CN4.C16 21.7,74.96 11.27,74.96 CN8.C16
  Bottom 0.152: v32.18,109.16 27.87,109.16 v27.75,109.29 | v122,41.58 118.56,41.58 v117.82,40.84 | v27.14,73.76 v25.66,73.76 v25.65,73.75
GND  (via drill 0.3, 0.35)
  Top 0.152: PKG4.58 99.62,71.97 v99.38,72.21
  Top 0.305: PKG1.106 65.9,101.58 v65.89,101.56 | PKG1.23 33.78,96.38 v33.76,96.4 | PKG1.26 38.05,94.42 v38.07,94.44 | PKG1.34 33.76,89.22 v33.74,89.24 | PKG1.40 v33.76,85.33 v33.75,85.33 | PKG1.18 v38.1,99.62 v38.11,99.62 | PKG1.4 37.58,108.72 v37.96,108.34 | PKG1.160 v39.33,116.28 v39.32,116.29 | PKG1.154 v43.23,116.28 v43.23,116.29 | PKG1.146 48.42,111.86 v48.4,111.84 | PKG1.143 v50.38,116.38 v50.37,116.38 | PKG1.124 62.73,112.38 v62.43,112.08 | PKG1.120 69.7,110.67 70.35,110.02 v70.35,109.08 | PKG1.114 70.31,106.78 v70.34,106.74 | PKG1.103 70.25,99.62 v70.29,99.67 | PKG1.98 70.28,96.38 v70.3,96.4 | PKG1.84 66.42,87.28 v66.09,87.61 | PKG1.80 v64.67,79.8 v64.68,79.79 | PKG1.74 60.77,79.83 v60.73,79.79 | PKG1.66 55.58,83.67 v56,84.1 | PKG1.63 53.62,79.72 v53.6,79.7 | PKG1.58 50.38,79.74 v50.33,79.7 | PKG1.44 41.27,83.58 v41.61,83.91 | PKG4.63 96.38,66.59 96.1,66.32 94.63,66.32 | PKG4.66 94.42,66.53 | 94.42,66.53 94.63,66.32 | 94.63,66.32 94.44,66.13 v94.44,65.86 94.42,65.87 94.42,66.53 | PKG4.84 83.56,62.73 v83.91,62.37 | PKG4.26 111.94,55.58 v111.92,55.59 | PKG4.23 116.22,53.62 v116.24,53.65 | PKG4.18 112.03,50.38 v112.02,50.39 | PKG4.4 112.56,41.27 v112.17,41.66 | PKG4.154 106.78,33.85 v106.74,33.82 | PKG4.160 v110.67,33.76 v110.67,33.75 | PKG4.143 v99.62,33.77 | PKG4.146 101.58,38.02 v101.67,38.12 | PKG4.124 87.28,37.56 v87.66,37.95 | PKG4.114 79.67,43.23 v79.63,43.27 | PKG4.103 79.81,50.38 v79.78,50.41 | PKG4.106 84.01,48.42 v84.03,48.41 | PKG4.98 79.83,53.62 v79.78,53.58 | PKG4.44 108.72,66.39 v108.41,66.08 | PKG4.40 116.31,64.67 v116.32,64.69 | PKG4.34 116.23,60.77 v116.28,60.73 | PKG4.120 80.34,39.33 79.59,40.07 v79.59,40.56
  Top 0.305: PKG4.80 v85.33,70.3 | PKG4.74 89.26,68.18 v89.26,70.31 | PKG4.138 96.38,33.7 v96.39,33.69 | PKG1.138 v53.62,116.65 v53.63,116.65
  pour Bottom (rank 2): -5,155 -5,-5 155,-5 155,155
PKG1/A_SOUT_CH1  (via drill 0.3)
  Top 0.152: PKG1.15 32.49,101.58 v32.18,101.88 | v27.47,101.89 27.79,102.22 27.79,108.38 27.14,109.03 27.14,109.54 27.42,109.82 27.42,111.32 28.35,112.25 28.35,114.05 35.95,121.65 44.64,121.65 45.29,122.3 47.1,122.3 48.31,121.09 54.43,121.09 55.36,122.02 55.86,122.02 56.51,121.37 63.69,121.37 64.49,122.17 66.66,122.17 67.38,122.89 67.38,130.88 CN3.A14 69.93,133.43 69.93,143.76 CN7.A14
  Bottom 0.152: v27.47,101.89 v27.48,101.88 v32.18,101.88
PKG1/A_SOUT_CH2  (via drill 0.3)
  Top 0.152: PKG1.55 48.42,78.69 48.23,78.5 v48.23,78.18 | v50.49,75.7 50.81,76.03 52.23,76.03 52.79,75.47 56.25,75.47 56.9,74.82 57.94,74.82 58.09,74.96 v73.92,74.96 | CN7.A18 80.08,143.77 80.08,133.42 CN3.A18 77.57,130.91 77.57,122.22 82.61,117.17 82.61,114.11 80.44,111.94 80.44,102.63 79.37,101.56 79.37,101.04 80.16,100.25 80.16,91.85 79.39,91.08 79.39,89.92 80.16,89.15 80.16,79.05 v76.08,74.96
  Bottom 0.152: v48.23,78.18 48.44,78.18 49.24,77.38 49.48,77.15 49.94,77.15 50.49,76.6 v50.49,75.7 | v76.08,74.96 v73.92,74.96
PKG1/A_SOUT_CH3  (via drill 0.3)
  Top 0.152: PKG1.95 71.59,94.42 v71.62,94.39 | v74.3,94.39 73.97,94.72 73.97,102.35 74.62,103 74.62,107.78 73.97,108.43 73.97,113.34 69.92,117.39 69.92,130.88 CN3.A15 72.46,133.42 72.46,143.77 CN7.A15
  Bottom 0.152: v71.62,94.39 v74.29,94.39 v74.3,94.39
PKG1/A_SOUT_CH4  (via drill 0.3)
  Top 0.152: PKG1.135 55.58,117.54 v55.61,117.57 | v55.61,121.41 55.94,121.09 63.81,121.09 64.61,121.89 68.02,121.89 68.65,122.53 CN3.C14
  Route15 0.152: CN7.C14 69.92,138.69 69.92,128.34 CN3.C14
  Bottom 0.152: v55.61,117.57 v55.61,121.41
PKG1/FR_CO  (via drill 0.3)
  Top 0.152: PKG1.1 v31.76,110.67 v31.75,110.67 | v28.87,110.67 29.19,110.34 29.19,99.1 28.54,98.45 28.54,97.25 28.91,96.88 28.91,93.21 28.26,92.56 28.26,91.36 28.63,90.99 28.63,65.62 28.54,65.53 28.54,63.04 29.16,62.42 29.16,48.25 29.16,48.13 29.16,35.15 36.79,27.52 64.47,27.52 v64.8,27.19 | v64.8,25.14 64.8,18.92 65.87,17.85 CN1.A20 67.38,16.58 67.38,6.23 CN5.A20
  Bottom 0.152: v31.75,110.67 v28.87,110.67 | v64.8,27.19 v64.8,25.14
PKG1/FR_CO_CH2/FR_CI_CH1  (via drill 0.3)
  Top 0.152: PKG1.41 39.33,77.88 v39.2,77.75 | v39.2,75.42 38.87,75.75 36.55,75.75 29.75,82.55 29.75,91.15 30.31,91.71 30.31,96.88 30.87,97.44 30.87,112.99 37.01,119.13 43.97,119.13 44.49,118.61 44.72,118.61 45.17,118.16 PKG1.151
  Bottom 0.152: v39.2,77.75 v39.2,75.42
PKG1/FR_CO_CH3/FR_CI_CH2  (via drill 0.3)
  Top 0.152: PKG1.81 v72.24,85.33 v72.25,85.32 | v74.58,85.32 74.25,84.99 74.25,82.55 67.45,75.75 58.78,75.75 58.22,76.31 53.14,76.31 52.58,76.87 37.01,76.87 30.87,83.01 30.87,90.69 31.35,91.17 PKG1.31
  Bottom 0.152: v72.25,85.32 v74.58,85.32
PKG1/FR_CO_CH4/FR_CI_CH3  (via drill 0.3)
